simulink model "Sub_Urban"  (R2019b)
settings: Solver=FixedStepAuto  StartTime=0.0  StopTime=3600*24  FixedStep=Tstep  MaxStep=1800  RelTol=1e-3
InitFcn:
  | load('network_parameters')
  | Vnom=400/sqrt(3);
  | Tstep=30*60;
  | MV_LV_transf=0;
StopFcn:
  | run('Simulink_Data.m')
undefined symbols (not defined in the file or in its folder): C_xlpe_185_90, D11, Delta, L_2x16mm, L_2x22mm, L_4x100mm, L_4x16mm, L_4x22mm, L_4x50mm, L_xlpe_185_90, LC, Line_length, R_2x16mm, R_2x22mm, R_4x100mm, R_4x16mm, R_4x22mm, R_4x50mm, R_xlpe_185_90, Source_Voltage
libraries: myLibrary x125, powerlib x89
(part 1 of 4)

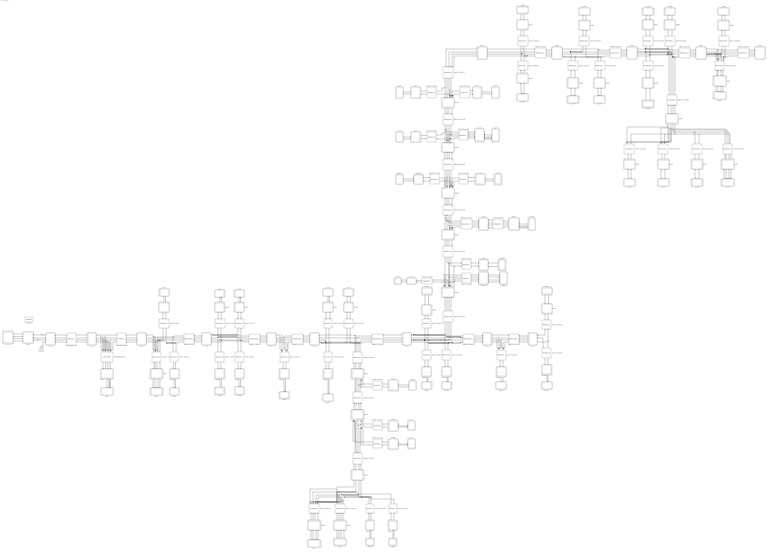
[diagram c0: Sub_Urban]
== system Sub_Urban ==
  100mm^2 Line 12 : powerlib/Elements/Mutual Inductance  LConnTagsString=a|b|c|L4  RConnTagsString=A|B|C|R4  TypeOfMutual=Generalized mutual inductance  NumberOfWindings=4  SelfImpedance1=[1.1 1.1e-03]  SelfImpedance2=[ 1.1 1.1e-03]  ThreeWindings=on  SelfImpedance3=[ 1.1 1.1e-03]  MutualImpedance=[1.0 1.0e-03]  InductanceMatrix=L_4x100mm*Line_length(13)  ResistanceMatrix=R_4x100mm*Line_length(13)  Measurements=None
  100mm^2 Line 14 : powerlib/Elements/Mutual Inductance  LConnTagsString=a|b|c|L4  RConnTagsString=A|B|C|R4  TypeOfMutual=Generalized mutual inductance  NumberOfWindings=4  SelfImpedance1=[1.1 1.1e-03]  SelfImpedance2=[ 1.1 1.1e-03]  ThreeWindings=on  SelfImpedance3=[ 1.1 1.1e-03]  MutualImpedance=[1.0 1.0e-03]  InductanceMatrix=L_4x100mm*Line_length(15)  ResistanceMatrix=R_4x100mm*Line_length(15)  Measurements=None
  100mm^2 Line 18 : powerlib/Elements/Mutual Inductance  LConnTagsString=a|b|c|L4  RConnTagsString=A|B|C|R4  TypeOfMutual=Generalized mutual inductance  NumberOfWindings=4  SelfImpedance1=[1.1 1.1e-03]  SelfImpedance2=[ 1.1 1.1e-03]  ThreeWindings=on  SelfImpedance3=[ 1.1 1.1e-03]  MutualImpedance=[1.0 1.0e-03]  InductanceMatrix=L_4x100mm*Line_length(19)  ResistanceMatrix=R_4x100mm*Line_length(19)  Measurements=None
  100mm^2 Line 20 : powerlib/Elements/Mutual Inductance  LConnTagsString=a|b|c|L4  RConnTagsString=A|B|C|R4  TypeOfMutual=Generalized mutual inductance  NumberOfWindings=4  SelfImpedance1=[1.1 1.1e-03]  SelfImpedance2=[ 1.1 1.1e-03]  ThreeWindings=on  SelfImpedance3=[ 1.1 1.1e-03]  MutualImpedance=[1.0 1.0e-03]  InductanceMatrix=L_4x100mm*Line_length(21)  ResistanceMatrix=R_4x100mm*Line_length(21)  Measurements=None
  100mm^2 Line 23 : powerlib/Elements/Mutual Inductance  LConnTagsString=a|b|c|L4  RConnTagsString=A|B|C|R4  TypeOfMutual=Generalized mutual inductance  NumberOfWindings=4  SelfImpedance1=[1.1 1.1e-03]  SelfImpedance2=[ 1.1 1.1e-03]  ThreeWindings=on  SelfImpedance3=[ 1.1 1.1e-03]  MutualImpedance=[1.0 1.0e-03]  InductanceMatrix=L_4x100mm*Line_length(24)  ResistanceMatrix=R_4x100mm*Line_length(24)  Measurements=None
  100mm^2 Line 28 : powerlib/Elements/Mutual Inductance  LConnTagsString=a|b|c|L4  RConnTagsString=A|B|C|R4  TypeOfMutual=Generalized mutual inductance  NumberOfWindings=4  SelfImpedance1=[1.1 1.1e-03]  SelfImpedance2=[ 1.1 1.1e-03]  ThreeWindings=on  SelfImpedance3=[ 1.1 1.1e-03]  MutualImpedance=[1.0 1.0e-03]  InductanceMatrix=L_4x100mm*Line_length(29)  ResistanceMatrix=R_4x100mm*Line_length(29)  Measurements=None
  100mm^2 Line 29 : powerlib/Elements/Mutual Inductance  LConnTagsString=a|b|c|L4  RConnTagsString=A|B|C|R4  TypeOfMutual=Generalized mutual inductance  NumberOfWindings=4  SelfImpedance1=[1.1 1.1e-03]  SelfImpedance2=[ 1.1 1.1e-03]  ThreeWindings=on  SelfImpedance3=[ 1.1 1.1e-03]  MutualImpedance=[1.0 1.0e-03]  InductanceMatrix=L_4x100mm*Line_length(30)  ResistanceMatrix=R_4x100mm*Line_length(30)  Measurements=None
  100mm^2 Line 31 : powerlib/Elements/Mutual Inductance  LConnTagsString=a|b|c|L4  RConnTagsString=A|B|C|R4  TypeOfMutual=Generalized mutual inductance  NumberOfWindings=4  SelfImpedance1=[1.1 1.1e-03]  SelfImpedance2=[ 1.1 1.1e-03]  ThreeWindings=on  SelfImpedance3=[ 1.1 1.1e-03]  MutualImpedance=[1.0 1.0e-03]  InductanceMatrix=L_4x100mm*Line_length(32)  ResistanceMatrix=R_4x100mm*Line_length(32)  Measurements=None
  100mm^2 Line 37 : powerlib/Elements/Mutual Inductance  LConnTagsString=a|b|c|L4  RConnTagsString=A|B|C|R4  TypeOfMutual=Generalized mutual inductance  NumberOfWindings=4  SelfImpedance1=[1.1 1.1e-03]  SelfImpedance2=[ 1.1 1.1e-03]  ThreeWindings=on  SelfImpedance3=[ 1.1 1.1e-03]  MutualImpedance=[1.0 1.0e-03]  InductanceMatrix=L_4x100mm*Line_length(38)  ResistanceMatrix=R_4x100mm*Line_length(38)  Measurements=None
  100mm^2 Line 41 : powerlib/Elements/Mutual Inductance  LConnTagsString=a|b|c|L4  RConnTagsString=A|B|C|R4  TypeOfMutual=Generalized mutual inductance  NumberOfWindings=4  SelfImpedance1=[1.1 1.1e-03]  SelfImpedance2=[ 1.1 1.1e-03]  ThreeWindings=on  SelfImpedance3=[ 1.1 1.1e-03]  MutualImpedance=[1.0 1.0e-03]  InductanceMatrix=L_4x100mm*Line_length(42)  ResistanceMatrix=R_4x100mm*Line_length(42)  Measurements=None
  100mm^2 Line 42 : powerlib/Elements/Mutual Inductance  LConnTagsString=a|b|c|L4  RConnTagsString=A|B|C|R4  TypeOfMutual=Generalized mutual inductance  NumberOfWindings=4  SelfImpedance1=[1.1 1.1e-03]  SelfImpedance2=[ 1.1 1.1e-03]  ThreeWindings=on  SelfImpedance3=[ 1.1 1.1e-03]  MutualImpedance=[1.0 1.0e-03]  InductanceMatrix=L_4x100mm*Line_length(43)  ResistanceMatrix=R_4x100mm*Line_length(43)  Measurements=None
  100mm^2 Line 44 : powerlib/Elements/Mutual Inductance  LConnTagsString=a|b|c|L4  RConnTagsString=A|B|C|R4  TypeOfMutual=Generalized mutual inductance  NumberOfWindings=4  SelfImpedance1=[1.1 1.1e-03]  SelfImpedance2=[ 1.1 1.1e-03]  ThreeWindings=on  SelfImpedance3=[ 1.1 1.1e-03]  MutualImpedance=[1.0 1.0e-03]  InductanceMatrix=L_4x100mm*Line_length(45)  ResistanceMatrix=R_4x100mm*Line_length(45)  Measurements=None
  100mm^2 Line 47 : powerlib/Elements/Mutual Inductance  LConnTagsString=a|b|c|L4  RConnTagsString=A|B|C|R4  TypeOfMutual=Generalized mutual inductance  NumberOfWindings=4  SelfImpedance1=[1.1 1.1e-03]  SelfImpedance2=[ 1.1 1.1e-03]  ThreeWindings=on  SelfImpedance3=[ 1.1 1.1e-03]  MutualImpedance=[1.0 1.0e-03]  InductanceMatrix=L_4x100mm*Line_length(48)  ResistanceMatrix=R_4x100mm*Line_length(48)  Measurements=None
  100mm^2 Line 50 : powerlib/Elements/Mutual Inductance  LConnTagsString=a|b|c|L4  RConnTagsString=A|B|C|R4  TypeOfMutual=Generalized mutual inductance  NumberOfWindings=4  SelfImpedance1=[1.1 1.1e-03]  SelfImpedance2=[ 1.1 1.1e-03]  ThreeWindings=on  SelfImpedance3=[ 1.1 1.1e-03]  MutualImpedance=[1.0 1.0e-03]  InductanceMatrix=L_4x100mm*Line_length(51)  ResistanceMatrix=R_4x100mm*Line_length(51)  Measurements=None
  100mm^2 Line 68 : powerlib/Elements/Mutual Inductance  LConnTagsString=a|b|c|L4  RConnTagsString=A|B|C|R4  TypeOfMutual=Generalized mutual inductance  NumberOfWindings=4  SelfImpedance1=[1.1 1.1e-03]  SelfImpedance2=[ 1.1 1.1e-03]  ThreeWindings=on  SelfImpedance3=[ 1.1 1.1e-03]  MutualImpedance=[1.0 1.0e-03]  InductanceMatrix=L_4x100mm*Line_length(69)  ResistanceMatrix=R_4x100mm*Line_length(69)  Measurements=None
  100mm^2 Line 7 : powerlib/Elements/Mutual Inductance  LConnTagsString=a|b|c|L4  RConnTagsString=A|B|C|R4  TypeOfMutual=Generalized mutual inductance  NumberOfWindings=4  SelfImpedance1=[1.1 1.1e-03]  SelfImpedance2=[ 1.1 1.1e-03]  ThreeWindings=on  SelfImpedance3=[ 1.1 1.1e-03]  MutualImpedance=[1.0 1.0e-03]  InductanceMatrix=L_4x100mm*Line_length(8)  ResistanceMatrix=R_4x100mm*Line_length(8)  Measurements=None
  16mm^2 Line 24 : powerlib/Elements/Mutual Inductance  LConnTagsString=a|b|c|L4  RConnTagsString=A|B|C|R4  TypeOfMutual=Generalized mutual inductance  NumberOfWindings=4  SelfImpedance1=[1.1 1.1e-03]  SelfImpedance2=[ 1.1 1.1e-03]  ThreeWindings=on  SelfImpedance3=[ 1.1 1.1e-03]  MutualImpedance=[1.0 1.0e-03]  InductanceMatrix=L_4x16mm*Line_length(25)  ResistanceMatrix=R_4x16mm*Line_length(25)  Measurements=None
  16mm^2 Line 25 : powerlib/Elements/Mutual Inductance  LConnTagsString=a|b|c|L4  RConnTagsString=A|B|C|R4  TypeOfMutual=Generalized mutual inductance  NumberOfWindings=4  SelfImpedance1=[1.1 1.1e-03]  SelfImpedance2=[ 1.1 1.1e-03]  ThreeWindings=on  SelfImpedance3=[ 1.1 1.1e-03]  MutualImpedance=[1.0 1.0e-03]  InductanceMatrix=L_4x16mm*Line_length(26)  ResistanceMatrix=R_4x16mm*Line_length(26)  Measurements=None
  16mm^2 Line 34 : powerlib/Elements/Mutual Inductance  LConnTagsString=a|b  RConnTagsString=A|B  TypeOfMutual=Generalized mutual inductance  NumberOfWindings=2  SelfImpedance1=[1.1 1.1e-03]  SelfImpedance2=[ 1.1 1.1e-03]  ThreeWindings=on  SelfImpedance3=[ 1.1 1.1e-03]  MutualImpedance=[1.0 1.0e-03]  InductanceMatrix=L_2x16mm*Line_length(35)  ResistanceMatrix=R_2x16mm*Line_length(35)  Measurements=None
  16mm^2 Line 62 : powerlib/Elements/Mutual Inductance  LConnTagsString=a|b|c|L4  RConnTagsString=A|B|C|R4  TypeOfMutual=Generalized mutual inductance  NumberOfWindings=4  SelfImpedance1=[1.1 1.1e-03]  SelfImpedance2=[ 1.1 1.1e-03]  ThreeWindings=on  SelfImpedance3=[ 1.1 1.1e-03]  MutualImpedance=[1.0 1.0e-03]  InductanceMatrix=L_4x16mm*Line_length(63)  ResistanceMatrix=R_4x16mm*Line_length(63)  Measurements=None
  16mm^2 Line 8 : powerlib/Elements/Mutual Inductance  LConnTagsString=a|b  RConnTagsString=A|B  TypeOfMutual=Generalized mutual inductance  NumberOfWindings=2  SelfImpedance1=[1.1 1.1e-03]  SelfImpedance2=[ 1.1 1.1e-03]  ThreeWindings=on  SelfImpedance3=[ 1.1 1.1e-03]  MutualImpedance=[1.0 1.0e-03]  InductanceMatrix=L_2x16mm*Line_length(9)  ResistanceMatrix=R_2x16mm*Line_length(9)  Measurements=None
  22mm^2 Line 10 : powerlib/Elements/Mutual Inductance  LConnTagsString=a|b  RConnTagsString=A|B  TypeOfMutual=Generalized mutual inductance  NumberOfWindings=2  SelfImpedance1=[1.1 1.1e-03]  SelfImpedance2=[ 1.1 1.1e-03]  ThreeWindings=on  SelfImpedance3=[ 1.1 1.1e-03]  MutualImpedance=[1.0 1.0e-03]  InductanceMatrix=L_2x22mm*Line_length(11)  ResistanceMatrix=R_2x22mm*Line_length(11)  Measurements=None
  22mm^2 Line 11 : powerlib/Elements/Mutual Inductance  LConnTagsString=a|b  RConnTagsString=A|B  TypeOfMutual=Generalized mutual inductance  NumberOfWindings=2  SelfImpedance1=[1.1 1.1e-03]  SelfImpedance2=[ 1.1 1.1e-03]  ThreeWindings=on  SelfImpedance3=[ 1.1 1.1e-03]  MutualImpedance=[1.0 1.0e-03]  InductanceMatrix=L_2x22mm*Line_length(12)  ResistanceMatrix=R_2x22mm*Line_length(12)  Measurements=None
  22mm^2 Line 13 : powerlib/Elements/Mutual Inductance  LConnTagsString=a|b  RConnTagsString=A|B  TypeOfMutual=Generalized mutual inductance  NumberOfWindings=2  SelfImpedance1=[1.1 1.1e-03]  SelfImpedance2=[ 1.1 1.1e-03]  ThreeWindings=on  SelfImpedance3=[ 1.1 1.1e-03]  MutualImpedance=[1.0 1.0e-03]  InductanceMatrix=L_2x22mm*Line_length(14)  ResistanceMatrix=R_2x22mm*Line_length(14)  Measurements=None
  22mm^2 Line 15 : powerlib/Elements/Mutual Inductance  LConnTagsString=a|b  RConnTagsString=A|B  TypeOfMutual=Generalized mutual inductance  NumberOfWindings=2  SelfImpedance1=[1.1 1.1e-03]  SelfImpedance2=[ 1.1 1.1e-03]  ThreeWindings=on  SelfImpedance3=[ 1.1 1.1e-03]  MutualImpedance=[1.0 1.0e-03]  InductanceMatrix=L_2x22mm*Line_length(16)  ResistanceMatrix=R_2x22mm*Line_length(16)  Measurements=None
  22mm^2 Line 16 : powerlib/Elements/Mutual Inductance  LConnTagsString=a|b  RConnTagsString=A|B  TypeOfMutual=Generalized mutual inductance  NumberOfWindings=2  SelfImpedance1=[1.1 1.1e-03]  SelfImpedance2=[ 1.1 1.1e-03]  ThreeWindings=on  SelfImpedance3=[ 1.1 1.1e-03]  MutualImpedance=[1.0 1.0e-03]  InductanceMatrix=L_2x22mm*Line_length(17)  ResistanceMatrix=R_2x22mm*Line_length(17)  Measurements=None
  22mm^2 Line 17 : powerlib/Elements/Mutual Inductance  LConnTagsString=a|b  RConnTagsString=A|B  TypeOfMutual=Generalized mutual inductance  NumberOfWindings=2  SelfImpedance1=[1.1 1.1e-03]  SelfImpedance2=[ 1.1 1.1e-03]  ThreeWindings=on  SelfImpedance3=[ 1.1 1.1e-03]  MutualImpedance=[1.0 1.0e-03]  InductanceMatrix=L_2x22mm*Line_length(18)  ResistanceMatrix=R_2x22mm*Line_length(18)  Measurements=None
  22mm^2 Line 19 : powerlib/Elements/Mutual Inductance  LConnTagsString=a|b  RConnTagsString=A|B  TypeOfMutual=Generalized mutual inductance  NumberOfWindings=2  SelfImpedance1=[1.1 1.1e-03]  SelfImpedance2=[ 1.1 1.1e-03]  ThreeWindings=on  SelfImpedance3=[ 1.1 1.1e-03]  MutualImpedance=[1.0 1.0e-03]  InductanceMatrix=L_2x22mm*Line_length(20)  ResistanceMatrix=R_2x22mm*Line_length(20)  Measurements=None
  22mm^2 Line 21 : powerlib/Elements/Mutual Inductance  LConnTagsString=a|b  RConnTagsString=A|B  TypeOfMutual=Generalized mutual inductance  NumberOfWindings=2  SelfImpedance1=[1.1 1.1e-03]  SelfImpedance2=[ 1.1 1.1e-03]  ThreeWindings=on  SelfImpedance3=[ 1.1 1.1e-03]  MutualImpedance=[1.0 1.0e-03]  InductanceMatrix=L_2x22mm*Line_length(22)  ResistanceMatrix=R_2x22mm*Line_length(22)  Measurements=None
  22mm^2 Line 22 : powerlib/Elements/Mutual Inductance  LConnTagsString=a|b  RConnTagsString=A|B  TypeOfMutual=Generalized mutual inductance  NumberOfWindings=2  SelfImpedance1=[1.1 1.1e-03]  SelfImpedance2=[ 1.1 1.1e-03]  ThreeWindings=on  SelfImpedance3=[ 1.1 1.1e-03]  MutualImpedance=[1.0 1.0e-03]  InductanceMatrix=L_2x22mm*Line_length(23)  ResistanceMatrix=R_2x22mm*Line_length(23)  Measurements=None
  22mm^2 Line 26 : powerlib/Elements/Mutual Inductance  LConnTagsString=a|b  RConnTagsString=A|B  TypeOfMutual=Generalized mutual inductance  NumberOfWindings=2  SelfImpedance1=[1.1 1.1e-03]  SelfImpedance2=[ 1.1 1.1e-03]  ThreeWindings=on  SelfImpedance3=[ 1.1 1.1e-03]  MutualImpedance=[1.0 1.0e-03]  InductanceMatrix=L_2x22mm*Line_length(27)  ResistanceMatrix=R_2x22mm*Line_length(27)  Measurements=None
  22mm^2 Line 27 : powerlib/Elements/Mutual Inductance  LConnTagsString=a|b  RConnTagsString=A|B  TypeOfMutual=Generalized mutual inductance  NumberOfWindings=2  SelfImpedance1=[1.1 1.1e-03]  SelfImpedance2=[ 1.1 1.1e-03]  ThreeWindings=on  SelfImpedance3=[ 1.1 1.1e-03]  MutualImpedance=[1.0 1.0e-03]  InductanceMatrix=L_2x22mm*Line_length(28)  ResistanceMatrix=R_2x22mm*Line_length(28)  Measurements=None
  22mm^2 Line 30 : powerlib/Elements/Mutual Inductance  LConnTagsString=a|b  RConnTagsString=A|B  TypeOfMutual=Generalized mutual inductance  NumberOfWindings=2  SelfImpedance1=[1.1 1.1e-03]  SelfImpedance2=[ 1.1 1.1e-03]  ThreeWindings=on  SelfImpedance3=[ 1.1 1.1e-03]  MutualImpedance=[1.0 1.0e-03]  InductanceMatrix=L_2x22mm*Line_length(31)  ResistanceMatrix=R_2x22mm*Line_length(31)  Measurements=None
  22mm^2 Line 32 : powerlib/Elements/Mutual Inductance  LConnTagsString=a|b  RConnTagsString=A|B  TypeOfMutual=Generalized mutual inductance  NumberOfWindings=2  SelfImpedance1=[1.1 1.1e-03]  SelfImpedance2=[ 1.1 1.1e-03]  ThreeWindings=on  SelfImpedance3=[ 1.1 1.1e-03]  MutualImpedance=[1.0 1.0e-03]  InductanceMatrix=L_2x22mm*Line_length(33)  ResistanceMatrix=R_2x22mm*Line_length(33)  Measurements=None
  22mm^2 Line 33 : powerlib/Elements/Mutual Inductance  LConnTagsString=a|b  RConnTagsString=A|B  TypeOfMutual=Generalized mutual inductance  NumberOfWindings=2  SelfImpedance1=[1.1 1.1e-03]  SelfImpedance2=[ 1.1 1.1e-03]  ThreeWindings=on  SelfImpedance3=[ 1.1 1.1e-03]  MutualImpedance=[1.0 1.0e-03]  InductanceMatrix=L_2x22mm*Line_length(34)  ResistanceMatrix=R_2x22mm*Line_length(34)  Measurements=None
  22mm^2 Line 35 : powerlib/Elements/Mutual Inductance  LConnTagsString=a|b  RConnTagsString=A|B  TypeOfMutual=Generalized mutual inductance  NumberOfWindings=2  SelfImpedance1=[1.1 1.1e-03]  SelfImpedance2=[ 1.1 1.1e-03]  ThreeWindings=on  SelfImpedance3=[ 1.1 1.1e-03]  MutualImpedance=[1.0 1.0e-03]  InductanceMatrix=L_2x22mm*Line_length(36)  ResistanceMatrix=R_2x22mm*Line_length(36)  Measurements=None
  22mm^2 Line 36 : powerlib/Elements/Mutual Inductance  LConnTagsString=a|b  RConnTagsString=A|B  TypeOfMutual=Generalized mutual inductance  NumberOfWindings=2  SelfImpedance1=[1.1 1.1e-03]  SelfImpedance2=[ 1.1 1.1e-03]  ThreeWindings=on  SelfImpedance3=[ 1.1 1.1e-03]  MutualImpedance=[1.0 1.0e-03]  InductanceMatrix=L_2x22mm*Line_length(37)  ResistanceMatrix=R_2x22mm*Line_length(37)  Measurements=None
  22mm^2 Line 38 : powerlib/Elements/Mutual Inductance  LConnTagsString=a|b|c|L4  RConnTagsString=A|B|C|R4  TypeOfMutual=Generalized mutual inductance  NumberOfWindings=4  SelfImpedance1=[1.1 1.1e-03]  SelfImpedance2=[ 1.1 1.1e-03]  ThreeWindings=on  SelfImpedance3=[ 1.1 1.1e-03]  MutualImpedance=[1.0 1.0e-03]  InductanceMatrix=L_4x22mm*Line_length(39)  ResistanceMatrix=R_4x22mm*Line_length(39)  Measurements=None
  22mm^2 Line 39 : powerlib/Elements/Mutual Inductance  LConnTagsString=a|b  RConnTagsString=A|B  TypeOfMutual=Generalized mutual inductance  NumberOfWindings=2  SelfImpedance1=[1.1 1.1e-03]  SelfImpedance2=[ 1.1 1.1e-03]  ThreeWindings=on  SelfImpedance3=[ 1.1 1.1e-03]  MutualImpedance=[1.0 1.0e-03]  InductanceMatrix=L_2x22mm*Line_length(40)  ResistanceMatrix=R_2x22mm*Line_length(40)  Measurements=None
  22mm^2 Line 4 : powerlib/Elements/Mutual Inductance  LConnTagsString=a|b|c|L4  RConnTagsString=A|B|C|R4  TypeOfMutual=Generalized mutual inductance  NumberOfWindings=4  SelfImpedance1=[1.1 1.1e-03]  SelfImpedance2=[ 1.1 1.1e-03]  ThreeWindings=on  SelfImpedance3=[ 1.1 1.1e-03]  MutualImpedance=[1.0 1.0e-03]  InductanceMatrix=L_4x22mm*Line_length(5)  ResistanceMatrix=R_4x22mm*Line_length(5)  Measurements=None
  22mm^2 Line 40 : powerlib/Elements/Mutual Inductance  LConnTagsString=a|b  RConnTagsString=A|B  TypeOfMutual=Generalized mutual inductance  NumberOfWindings=2  SelfImpedance1=[1.1 1.1e-03]  SelfImpedance2=[ 1.1 1.1e-03]  ThreeWindings=on  SelfImpedance3=[ 1.1 1.1e-03]  MutualImpedance=[1.0 1.0e-03]  InductanceMatrix=L_2x22mm*Line_length(41)  ResistanceMatrix=R_2x22mm*Line_length(41)  Measurements=None
  22mm^2 Line 43 : powerlib/Elements/Mutual Inductance  LConnTagsString=a|b|c|L4  RConnTagsString=A|B|C|R4  TypeOfMutual=Generalized mutual inductance  NumberOfWindings=4  SelfImpedance1=[1.1 1.1e-03]  SelfImpedance2=[ 1.1 1.1e-03]  ThreeWindings=on  SelfImpedance3=[ 1.1 1.1e-03]  MutualImpedance=[1.0 1.0e-03]  InductanceMatrix=L_4x22mm*Line_length(44)  ResistanceMatrix=R_4x22mm*Line_length(44)  Measurements=None
  22mm^2 Line 45 : powerlib/Elements/Mutual Inductance  LConnTagsString=a|b  RConnTagsString=A|B  TypeOfMutual=Generalized mutual inductance  NumberOfWindings=2  SelfImpedance1=[1.1 1.1e-03]  SelfImpedance2=[ 1.1 1.1e-03]  ThreeWindings=on  SelfImpedance3=[ 1.1 1.1e-03]  MutualImpedance=[1.0 1.0e-03]  InductanceMatrix=L_2x22mm*Line_length(46)  ResistanceMatrix=R_2x22mm*Line_length(46)  Measurements=None
  22mm^2 Line 46 : powerlib/Elements/Mutual Inductance  LConnTagsString=a|b  RConnTagsString=A|B  TypeOfMutual=Generalized mutual inductance  NumberOfWindings=2  SelfImpedance1=[1.1 1.1e-03]  SelfImpedance2=[ 1.1 1.1e-03]  ThreeWindings=on  SelfImpedance3=[ 1.1 1.1e-03]  MutualImpedance=[1.0 1.0e-03]  InductanceMatrix=L_2x22mm*Line_length(47)  ResistanceMatrix=R_2x22mm*Line_length(47)  Measurements=None
  22mm^2 Line 48 : powerlib/Elements/Mutual Inductance  LConnTagsString=a|b|c|L4  RConnTagsString=A|B|C|R4  TypeOfMutual=Generalized mutual inductance  NumberOfWindings=4  SelfImpedance1=[1.1 1.1e-03]  SelfImpedance2=[ 1.1 1.1e-03]  ThreeWindings=on  SelfImpedance3=[ 1.1 1.1e-03]  MutualImpedance=[1.0 1.0e-03]  InductanceMatrix=L_4x22mm*Line_length(49)  ResistanceMatrix=R_4x22mm*Line_length(49)  Measurements=None
  22mm^2 Line 49 : powerlib/Elements/Mutual Inductance  LConnTagsString=a|b  RConnTagsString=A|B  TypeOfMutual=Generalized mutual inductance  NumberOfWindings=2  SelfImpedance1=[1.1 1.1e-03]  SelfImpedance2=[ 1.1 1.1e-03]  ThreeWindings=on  SelfImpedance3=[ 1.1 1.1e-03]  MutualImpedance=[1.0 1.0e-03]  InductanceMatrix=L_2x22mm*Line_length(50)  ResistanceMatrix=R_2x22mm*Line_length(50)  Measurements=None
  22mm^2 Line 5 : powerlib/Elements/Mutual Inductance  LConnTagsString=a|b  RConnTagsString=A|B  TypeOfMutual=Generalized mutual inductance  NumberOfWindings=2  SelfImpedance1=[1.1 1.1e-03]  SelfImpedance2=[ 1.1 1.1e-03]  ThreeWindings=on  SelfImpedance3=[ 1.1 1.1e-03]  MutualImpedance=[1.0 1.0e-03]  InductanceMatrix=L_2x22mm*Line_length(6)  ResistanceMatrix=R_2x22mm*Line_length(6)  Measurements=None
  22mm^2 Line 51 : powerlib/Elements/Mutual Inductance  LConnTagsString=a|b  RConnTagsString=A|B  TypeOfMutual=Generalized mutual inductance  NumberOfWindings=2  SelfImpedance1=[1.1 1.1e-03]  SelfImpedance2=[ 1.1 1.1e-03]  ThreeWindings=on  SelfImpedance3=[ 1.1 1.1e-03]  MutualImpedance=[1.0 1.0e-03]  InductanceMatrix=L_2x22mm*Line_length(52)  ResistanceMatrix=R_2x22mm*Line_length(52)  Measurements=None
  22mm^2 Line 52 : powerlib/Elements/Mutual Inductance  LConnTagsString=a|b  RConnTagsString=A|B  TypeOfMutual=Generalized mutual inductance  NumberOfWindings=2  SelfImpedance1=[1.1 1.1e-03]  SelfImpedance2=[ 1.1 1.1e-03]  ThreeWindings=on  SelfImpedance3=[ 1.1 1.1e-03]  MutualImpedance=[1.0 1.0e-03]  InductanceMatrix=L_2x22mm*Line_length(53)  ResistanceMatrix=R_2x22mm*Line_length(53)  Measurements=None
  22mm^2 Line 54 : powerlib/Elements/Mutual Inductance  LConnTagsString=a|b  RConnTagsString=A|B  TypeOfMutual=Generalized mutual inductance  NumberOfWindings=2  SelfImpedance1=[1.1 1.1e-03]  SelfImpedance2=[ 1.1 1.1e-03]  ThreeWindings=on  SelfImpedance3=[ 1.1 1.1e-03]  MutualImpedance=[1.0 1.0e-03]  InductanceMatrix=L_2x22mm*Line_length(55)  ResistanceMatrix=R_2x22mm*Line_length(55)  Measurements=None
  22mm^2 Line 55 : powerlib/Elements/Mutual Inductance  LConnTagsString=a|b  RConnTagsString=A|B  TypeOfMutual=Generalized mutual inductance  NumberOfWindings=2  SelfImpedance1=[1.1 1.1e-03]  SelfImpedance2=[ 1.1 1.1e-03]  ThreeWindings=on  SelfImpedance3=[ 1.1 1.1e-03]  MutualImpedance=[1.0 1.0e-03]  InductanceMatrix=L_2x22mm*Line_length(56)  ResistanceMatrix=R_2x22mm*Line_length(56)  Measurements=None
  22mm^2 Line 57 : powerlib/Elements/Mutual Inductance  LConnTagsString=a|b  RConnTagsString=A|B  TypeOfMutual=Generalized mutual inductance  NumberOfWindings=2  SelfImpedance1=[1.1 1.1e-03]  SelfImpedance2=[ 1.1 1.1e-03]  ThreeWindings=on  SelfImpedance3=[ 1.1 1.1e-03]  MutualImpedance=[1.0 1.0e-03]  InductanceMatrix=L_2x22mm*Line_length(58)  ResistanceMatrix=R_2x22mm*Line_length(58)  Measurements=None
  22mm^2 Line 58 : powerlib/Elements/Mutual Inductance  LConnTagsString=a|b  RConnTagsString=A|B  TypeOfMutual=Generalized mutual inductance  NumberOfWindings=2  SelfImpedance1=[1.1 1.1e-03]  SelfImpedance2=[ 1.1 1.1e-03]  ThreeWindings=on  SelfImpedance3=[ 1.1 1.1e-03]  MutualImpedance=[1.0 1.0e-03]  InductanceMatrix=L_2x22mm*Line_length(59)  ResistanceMatrix=R_2x22mm*Line_length(59)  Measurements=None
  22mm^2 Line 59 : powerlib/Elements/Mutual Inductance  LConnTagsString=a|b  RConnTagsString=A|B  TypeOfMutual=Generalized mutual inductance  NumberOfWindings=2  SelfImpedance1=[1.1 1.1e-03]  SelfImpedance2=[ 1.1 1.1e-03]  ThreeWindings=on  SelfImpedance3=[ 1.1 1.1e-03]  MutualImpedance=[1.0 1.0e-03]  InductanceMatrix=L_2x22mm*Line_length(60)  ResistanceMatrix=R_2x22mm*Line_length(60)  Measurements=None
  22mm^2 Line 6 : powerlib/Elements/Mutual Inductance  LConnTagsString=a|b  RConnTagsString=A|B  TypeOfMutual=Generalized mutual inductance  NumberOfWindings=2  SelfImpedance1=[1.1 1.1e-03]  SelfImpedance2=[ 1.1 1.1e-03]  ThreeWindings=on  SelfImpedance3=[ 1.1 1.1e-03]  MutualImpedance=[1.0 1.0e-03]  InductanceMatrix=L_2x22mm*Line_length(7)  ResistanceMatrix=R_2x22mm*Line_length(7)  Measurements=None
  22mm^2 Line 63 : powerlib/Elements/Mutual Inductance  LConnTagsString=a|b  RConnTagsString=A|B  TypeOfMutual=Generalized mutual inductance  NumberOfWindings=2  SelfImpedance1=[1.1 1.1e-03]  SelfImpedance2=[ 1.1 1.1e-03]  ThreeWindings=on  SelfImpedance3=[ 1.1 1.1e-03]  MutualImpedance=[1.0 1.0e-03]  InductanceMatrix=L_2x22mm*Line_length(64)  ResistanceMatrix=R_2x22mm*Line_length(64)  Measurements=None
  22mm^2 Line 65 : powerlib/Elements/Mutual Inductance  LConnTagsString=a|b  RConnTagsString=A|B  TypeOfMutual=Generalized mutual inductance  NumberOfWindings=2  SelfImpedance1=[1.1 1.1e-03]  SelfImpedance2=[ 1.1 1.1e-03]  ThreeWindings=on  SelfImpedance3=[ 1.1 1.1e-03]  MutualImpedance=[1.0 1.0e-03]  InductanceMatrix=L_2x22mm*Line_length(66)  ResistanceMatrix=R_2x22mm*Line_length(66)  Measurements=None
  22mm^2 Line 66 : powerlib/Elements/Mutual Inductance  LConnTagsString=a|b  RConnTagsString=A|B  TypeOfMutual=Generalized mutual inductance  NumberOfWindings=2  SelfImpedance1=[1.1 1.1e-03]  SelfImpedance2=[ 1.1 1.1e-03]  ThreeWindings=on  SelfImpedance3=[ 1.1 1.1e-03]  MutualImpedance=[1.0 1.0e-03]  InductanceMatrix=L_2x22mm*Line_length(67)  ResistanceMatrix=R_2x22mm*Line_length(67)  Measurements=None
  22mm^2 Line 67 : powerlib/Elements/Mutual Inductance  LConnTagsString=a|b  RConnTagsString=A|B  TypeOfMutual=Generalized mutual inductance  NumberOfWindings=2  SelfImpedance1=[1.1 1.1e-03]  SelfImpedance2=[ 1.1 1.1e-03]  ThreeWindings=on  SelfImpedance3=[ 1.1 1.1e-03]  MutualImpedance=[1.0 1.0e-03]  InductanceMatrix=L_2x22mm*Line_length(68)  ResistanceMatrix=R_2x22mm*Line_length(68)  Measurements=None
  22mm^2 Line 69 : powerlib/Elements/Mutual Inductance  LConnTagsString=a|b  RConnTagsString=A|B  TypeOfMutual=Generalized mutual inductance  NumberOfWindings=2  SelfImpedance1=[1.1 1.1e-03]  SelfImpedance2=[ 1.1 1.1e-03]  ThreeWindings=on  SelfImpedance3=[ 1.1 1.1e-03]  MutualImpedance=[1.0 1.0e-03]  InductanceMatrix=L_2x22mm*Line_length(70)  ResistanceMatrix=R_2x22mm*Line_length(70)  Measurements=None
  22mm^2 Line 70 : powerlib/Elements/Mutual Inductance  LConnTagsString=a|b  RConnTagsString=A|B  TypeOfMutual=Generalized mutual inductance  NumberOfWindings=2  SelfImpedance1=[1.1 1.1e-03]  SelfImpedance2=[ 1.1 1.1e-03]  ThreeWindings=on  SelfImpedance3=[ 1.1 1.1e-03]  MutualImpedance=[1.0 1.0e-03]  InductanceMatrix=L_2x22mm*Line_length(71)  ResistanceMatrix=R_2x22mm*Line_length(71)  Measurements=None
  22mm^2 Line 71 : powerlib/Elements/Mutual Inductance  LConnTagsString=a|b  RConnTagsString=A|B  TypeOfMutual=Generalized mutual inductance  NumberOfWindings=2  SelfImpedance1=[1.1 1.1e-03]  SelfImpedance2=[ 1.1 1.1e-03]  ThreeWindings=on  SelfImpedance3=[ 1.1 1.1e-03]  MutualImpedance=[1.0 1.0e-03]  InductanceMatrix=L_2x22mm*Line_length(72)  ResistanceMatrix=R_2x22mm*Line_length(72)  Measurements=None
  22mm^2 Line 72 : powerlib/Elements/Mutual Inductance  LConnTagsString=a|b|c|L4  RConnTagsString=A|B|C|R4  TypeOfMutual=Generalized mutual inductance  NumberOfWindings=4  SelfImpedance1=[1.1 1.1e-03]  SelfImpedance2=[ 1.1 1.1e-03]  ThreeWindings=on  SelfImpedance3=[ 1.1 1.1e-03]  MutualImpedance=[1.0 1.0e-03]  InductanceMatrix=L_4x22mm*Line_length(73)  ResistanceMatrix=R_4x22mm*Line_length(73)  Measurements=None
  22mm^2 Line 9 : powerlib/Elements/Mutual Inductance  LConnTagsString=a|b  RConnTagsString=A|B  TypeOfMutual=Generalized mutual inductance  NumberOfWindings=2  SelfImpedance1=[1.1 1.1e-03]  SelfImpedance2=[ 1.1 1.1e-03]  ThreeWindings=on  SelfImpedance3=[ 1.1 1.1e-03]  MutualImpedance=[1.0 1.0e-03]  InductanceMatrix=L_2x22mm*Line_length(10)  ResistanceMatrix=R_2x22mm*Line_length(10)  Measurements=None
  50mm^2 Line 53 : powerlib/Elements/Mutual Inductance  LConnTagsString=a|b|c|L4  RConnTagsString=A|B|C|R4  TypeOfMutual=Generalized mutual inductance  NumberOfWindings=4  SelfImpedance1=[1.1 1.1e-03]  SelfImpedance2=[ 1.1 1.1e-03]  ThreeWindings=on  SelfImpedance3=[ 1.1 1.1e-03]  MutualImpedance=[1.0 1.0e-03]  InductanceMatrix=L_4x50mm*Line_length(54)  ResistanceMatrix=R_4x50mm*Line_length(54)  Measurements=None
  50mm^2 Line 56 : powerlib/Elements/Mutual Inductance  LConnTagsString=a|b|c|L4  RConnTagsString=A|B|C|R4  TypeOfMutual=Generalized mutual inductance  NumberOfWindings=4  SelfImpedance1=[1.1 1.1e-03]  SelfImpedance2=[ 1.1 1.1e-03]  ThreeWindings=on  SelfImpedance3=[ 1.1 1.1e-03]  MutualImpedance=[1.0 1.0e-03]  InductanceMatrix=L_4x50mm*Line_length(57)  ResistanceMatrix=R_4x50mm*Line_length(57)  Measurements=None
  50mm^2 Line 60 : powerlib/Elements/Mutual Inductance  LConnTagsString=a|b|c|L4  RConnTagsString=A|B|C|R4  TypeOfMutual=Generalized mutual inductance  NumberOfWindings=4  SelfImpedance1=[1.1 1.1e-03]  SelfImpedance2=[ 1.1 1.1e-03]  ThreeWindings=on  SelfImpedance3=[ 1.1 1.1e-03]  MutualImpedance=[1.0 1.0e-03]  InductanceMatrix=L_4x50mm*Line_length(61)  ResistanceMatrix=R_4x50mm*Line_length(61)  Measurements=None
  50mm^2 Line 61 : powerlib/Elements/Mutual Inductance  LConnTagsString=a|b|c|L4  RConnTagsString=A|B|C|R4  TypeOfMutual=Generalized mutual inductance  NumberOfWindings=4  SelfImpedance1=[1.1 1.1e-03]  SelfImpedance2=[ 1.1 1.1e-03]  ThreeWindings=on  SelfImpedance3=[ 1.1 1.1e-03]  MutualImpedance=[1.0 1.0e-03]  InductanceMatrix=L_4x50mm*Line_length(62)  ResistanceMatrix=R_4x50mm*Line_length(62)  Measurements=None
  50mm^2 Line 64 : powerlib/Elements/Mutual Inductance  LConnTagsString=a|b|c|L4  RConnTagsString=A|B|C|R4  TypeOfMutual=Generalized mutual inductance  NumberOfWindings=4  SelfImpedance1=[1.1 1.1e-03]  SelfImpedance2=[ 1.1 1.1e-03]  ThreeWindings=on  SelfImpedance3=[ 1.1 1.1e-03]  MutualImpedance=[1.0 1.0e-03]  InductanceMatrix=L_4x50mm*Line_length(65)  ResistanceMatrix=R_4x50mm*Line_length(65)  Measurements=None
  Bus1 : Subsystem
  Bus10 : Subsystem  mask{Ph=3, Bus=10, Load=5}
      mask prompts: Ph "Phase [A=1, B=2, C=3]"; Bus "Bus Number"; Load "Load Number"
      mask init:
      | data_V=sprintf('Bus%d',Bus);
      | set_param([gcb '/To Workspace V'],'VariableName',data_V);
      | 
      | data_I=sprintf('I%d',Bus);
      | set_param([gcb '/To Workspace I'],'VariableName',data_I);
      | 
      | data_L=sprintf('Load%d',Load);
      | set_param([gcb '/To Workspace L'],'VariableName',data_L)
  Bus11 : Subsystem  mask{Ph=2, Bus=11, Load=6}
      mask prompts: Ph "Phase [A=1, B=2, C=3]"; Bus "Bus Number"; Load "Load Number"
      mask init:
      | data_V=sprintf('Bus%d',Bus);
      | set_param([gcb '/To Workspace V'],'VariableName',data_V);
      | 
      | data_I=sprintf('I%d',Bus);
      | set_param([gcb '/To Workspace I'],'VariableName',data_I);
      | 
      | data_L=sprintf('Load%d',Load);
      | set_param([gcb '/To Workspace L'],'VariableName',data_L)
  Bus12 : Subsystem  mask{Ph=2, Bus=12, Load=7}
      mask prompts: Ph "Phase [A=1, B=2, C=3]"; Bus "Bus Number"; Load "Load Number"
      mask init:
      | data_V=sprintf('Bus%d',Bus);
      | set_param([gcb '/To Workspace V'],'VariableName',data_V);
      | 
      | data_I=sprintf('I%d',Bus);
      | set_param([gcb '/To Workspace I'],'VariableName',data_I);
      | 
      | data_L=sprintf('Load%d',Load);
      | set_param([gcb '/To Workspace L'],'VariableName',data_L)
  Bus13 : Subsystem  mask{Ph=1, Bus=13, Load=8}
      mask prompts: Ph "Phase [A=1, B=2, C=3]"; Bus "Bus Number"; Load "Load Number"
      mask init:
      | data_V=sprintf('Bus%d',Bus);
      | set_param([gcb '/To Workspace V'],'VariableName',data_V);
      | 
      | data_I=sprintf('I%d',Bus);
      | set_param([gcb '/To Workspace I'],'VariableName',data_I);
      | 
      | data_L=sprintf('Load%d',Load);
      | set_param([gcb '/To Workspace L'],'VariableName',data_L)
  Bus14 : Subsystem  mask{Bus=14}
      mask prompts: Bus "Bus Number"
      mask init:
      | data_V=sprintf('Bus%d',Bus);
      | set_param([gcb '/To Workspace V'],'VariableName',data_V);
      | 
      | data_I=sprintf('I%d',Bus);
      | set_param([gcb '/To Workspace I'],'VariableName',data_I);
  Bus15 : Subsystem  mask{Ph=1, Bus=15, Load=9}
      mask prompts: Ph "Phase [A=1, B=2, C=3]"; Bus "Bus Number"; Load "Load Number"
      mask init:
      | data_V=sprintf('Bus%d',Bus);
      | set_param([gcb '/To Workspace V'],'VariableName',data_V);
      | 
      | data_I=sprintf('I%d',Bus);
      | set_param([gcb '/To Workspace I'],'VariableName',data_I);
      | 
      | data_L=sprintf('Load%d',Load);
      | set_param([gcb '/To Workspace L'],'VariableName',data_L)
  Bus16 : Subsystem  mask{Bus=16}
      mask prompts: Bus "Bus Number"
      mask init:
      | data_V=sprintf('Bus%d',Bus);
      | set_param([gcb '/To Workspace V'],'VariableName',data_V);
      | 
      | data_I=sprintf('I%d',Bus);
      | set_param([gcb '/To Workspace I'],'VariableName',data_I);
  Bus17 : Subsystem  mask{Ph=3, Bus=17, Load=10}
      mask prompts: Ph "Phase [A=1, B=2, C=3]"; Bus "Bus Number"; Load "Load Number"
      mask init:
      | data_V=sprintf('Bus%d',Bus);
      | set_param([gcb '/To Workspace V'],'VariableName',data_V);
      | 
      | data_I=sprintf('I%d',Bus);
      | set_param([gcb '/To Workspace I'],'VariableName',data_I);
      | 
      | data_L=sprintf('Load%d',Load);
      | set_param([gcb '/To Workspace L'],'VariableName',data_L)
  Bus18 : Subsystem  mask{Ph=3, Bus=18, Load=11}
      mask prompts: Ph "Phase [A=1, B=2, C=3]"; Bus "Bus Number"; Load "Load Number"
      mask init:
      | data_V=sprintf('Bus%d',Bus);
      | set_param([gcb '/To Workspace V'],'VariableName',data_V);
      | 
      | data_I=sprintf('I%d',Bus);
      | set_param([gcb '/To Workspace I'],'VariableName',data_I);
      | 
      | data_L=sprintf('Load%d',Load);
      | set_param([gcb '/To Workspace L'],'VariableName',data_L)
  Bus19 : Subsystem  mask{Ph=3, Bus=19, Load=12}
      mask prompts: Ph "Phase [A=1, B=2, C=3]"; Bus "Bus Number"; Load "Load Number"
      mask init:
      | data_V=sprintf('Bus%d',Bus);
      | set_param([gcb '/To Workspace V'],'VariableName',data_V);
      | 
      | data_I=sprintf('I%d',Bus);
      | set_param([gcb '/To Workspace I'],'VariableName',data_I);
      | 
      | data_L=sprintf('Load%d',Load);
      | set_param([gcb '/To Workspace L'],'VariableName',data_L)
  Bus2 : Subsystem  mask{Bus=2}
      mask prompts: Bus "Bus Number"
      mask init:
      | data_V=sprintf('Bus%d',Bus);
      | set_param([gcb '/To Workspace V'],'VariableName',data_V);
      | 
      | data_I=sprintf('I%d',Bus);
      | set_param([gcb '/To Workspace I'],'VariableName',data_I);
  Bus20 : Subsystem  mask{Bus=20}
      mask prompts: Bus "Bus Number"
      mask init:
      | data_V=sprintf('Bus%d',Bus);
      | set_param([gcb '/To Workspace V'],'VariableName',data_V);
      | 
      | data_I=sprintf('I%d',Bus);
      | set_param([gcb '/To Workspace I'],'VariableName',data_I);
  Bus21 : Subsystem  mask{Ph=3, Bus=21, Load=13}
      mask prompts: Ph "Phase [A=1, B=2, C=3]"; Bus "Bus Number"; Load "Load Number"
      mask init:
      | data_V=sprintf('Bus%d',Bus);
      | set_param([gcb '/To Workspace V'],'VariableName',data_V);
      | 
      | data_I=sprintf('I%d',Bus);
      | set_param([gcb '/To Workspace I'],'VariableName',data_I);
      | 
      | data_L=sprintf('Load%d',Load);
      | set_param([gcb '/To Workspace L'],'VariableName',data_L)
  Bus22 : Subsystem  mask{Bus=22}
      mask prompts: Bus "Bus Number"
      mask init:
      | data_V=sprintf('Bus%d',Bus);
      | set_param([gcb '/To Workspace V'],'VariableName',data_V);
      | 
      | data_I=sprintf('I%d',Bus);
      | set_param([gcb '/To Workspace I'],'VariableName',data_I);
  Bus23 : Subsystem  mask{Ph=3, Bus=23, Load=14}
      mask prompts: Ph "Phase [A=1, B=2, C=3]"; Bus "Bus Number"; Load "Load Number"
      mask init:
      | data_V=sprintf('Bus%d',Bus);
      | set_param([gcb '/To Workspace V'],'VariableName',data_V);
      | 
      | data_I=sprintf('I%d',Bus);
      | set_param([gcb '/To Workspace I'],'VariableName',data_I);
      | 
      | data_L=sprintf('Load%d',Load);
      | set_param([gcb '/To Workspace L'],'VariableName',data_L)
  Bus24 : Subsystem  mask{Ph=1, Bus=24, Load=15}
      mask prompts: Ph "Phase [A=1, B=2, C=3]"; Bus "Bus Number"; Load "Load Number"
      mask init:
      | data_V=sprintf('Bus%d',Bus);
      | set_param([gcb '/To Workspace V'],'VariableName',data_V);
      | 
      | data_I=sprintf('I%d',Bus);
      | set_param([gcb '/To Workspace I'],'VariableName',data_I);
      | 
      | data_L=sprintf('Load%d',Load);
      | set_param([gcb '/To Workspace L'],'VariableName',data_L)
  Bus25 : Subsystem  mask{Bus=25}
      mask prompts: Bus "Bus Number"
      mask init:
      | data_V=sprintf('Bus%d',Bus);
      | set_param([gcb '/To Workspace V'],'VariableName',data_V);
      | 
      | data_I=sprintf('I%d',Bus);
      | set_param([gcb '/To Workspace I'],'VariableName',data_I);
  Bus26 : Subsystem  mask{Bus=26, Load=16}
      mask prompts: Bus "Bus Number"; Load "Load Number"
      mask init:
      | data_V=sprintf('Bus%d',Bus);
      | set_param([gcb '/To Workspace V'],'VariableName',data_V);
      | 
      | data_I=sprintf('I%d',Bus);
      | set_param([gcb '/To Workspace I'],'VariableName',data_I);
      | 
      | data_L=sprintf('Load%d',Load);
      | set_param([gcb '/To Workspace L'],'VariableName',data_L)
  Bus27 : Subsystem  mask{Bus=27, Load=17}
      mask prompts: Bus "Bus Number"; Load "Load Number"
      mask init:
      | data_V=sprintf('Bus%d',Bus);
      | set_param([gcb '/To Workspace V'],'VariableName',data_V);
      | 
      | data_I=sprintf('I%d',Bus);
      | set_param([gcb '/To Workspace I'],'VariableName',data_I);
      | 
      | data_L=sprintf('Load%d',Load);
      | set_param([gcb '/To Workspace L'],'VariableName',data_L)
  Bus28 : Subsystem  mask{Ph=3, Bus=28, Load=18}
      mask prompts: Ph "Phase [A=1, B=2, C=3]"; Bus "Bus Number"; Load "Load Number"
      mask init:
      | data_V=sprintf('Bus%d',Bus);
      | set_param([gcb '/To Workspace V'],'VariableName',data_V);
      | 
      | data_I=sprintf('I%d',Bus);
      | set_param([gcb '/To Workspace I'],'VariableName',data_I);
      | 
      | data_L=sprintf('Load%d',Load);
      | set_param([gcb '/To Workspace L'],'VariableName',data_L)
  Bus29 : Subsystem  mask{Ph=2, Bus=29, Load=19}
      mask prompts: Ph "Phase [A=1, B=2, C=3]"; Bus "Bus Number"; Load "Load Number"
      mask init:
      | data_V=sprintf('Bus%d',Bus);
      | set_param([gcb '/To Workspace V'],'VariableName',data_V);
      | 
      | data_I=sprintf('I%d',Bus);
      | set_param([gcb '/To Workspace I'],'VariableName',data_I);
      | 
      | data_L=sprintf('Load%d',Load);
      | set_param([gcb '/To Workspace L'],'VariableName',data_L)
  Bus3 : Subsystem  mask{Bus=3}
      mask prompts: Bus "Bus Number"
      mask init:
      | data_V=sprintf('Bus%d',Bus);
      | set_param([gcb '/To Workspace V'],'VariableName',data_V);
      | 
      | data_I=sprintf('I%d',Bus);
      | set_param([gcb '/To Workspace I'],'VariableName',data_I);
  Bus30 : Subsystem  mask{Bus=30}
      mask prompts: Bus "Bus Number"
      mask init:
      | data_V=sprintf('Bus%d',Bus);
      | set_param([gcb '/To Workspace V'],'VariableName',data_V);
      | 
      | data_I=sprintf('I%d',Bus);
      | set_param([gcb '/To Workspace I'],'VariableName',data_I);
  Bus31 : Subsystem  mask{Bus=31}
      mask prompts: Bus "Bus Number"
      mask init:
      | data_V=sprintf('Bus%d',Bus);
      | set_param([gcb '/To Workspace V'],'VariableName',data_V);
      | 
      | data_I=sprintf('I%d',Bus);
      | set_param([gcb '/To Workspace I'],'VariableName',data_I);
  Bus32 : Subsystem  mask{Ph=2, Bus=32, Load=20}
      mask prompts: Ph "Phase [A=1, B=2, C=3]"; Bus "Bus Number"; Load "Load Number"
      mask init:
      | data_V=sprintf('Bus%d',Bus);
      | set_param([gcb '/To Workspace V'],'VariableName',data_V);
      | 
      | data_I=sprintf('I%d',Bus);
      | set_param([gcb '/To Workspace I'],'VariableName',data_I);
      | 
      | data_L=sprintf('Load%d',Load);
      | set_param([gcb '/To Workspace L'],'VariableName',data_L)
  Bus33 : Subsystem  mask{Bus=33}
      mask prompts: Bus "Bus Number"
      mask init:
      | data_V=sprintf('Bus%d',Bus);
      | set_param([gcb '/To Workspace V'],'VariableName',data_V);
      | 
      | data_I=sprintf('I%d',Bus);
      | set_param([gcb '/To Workspace I'],'VariableName',data_I);
  Bus34 : Subsystem  mask{Ph=2, Bus=34, Load=21}
      mask prompts: Ph "Phase [A=1, B=2, C=3]"; Bus "Bus Number"; Load "Load Number"
      mask init:
      | data_V=sprintf('Bus%d',Bus);
      | set_param([gcb '/To Workspace V'],'VariableName',data_V);
      | 
      | data_I=sprintf('I%d',Bus);
      | set_param([gcb '/To Workspace I'],'VariableName',data_I);
      | 
      | data_L=sprintf('Load%d',Load);
      | set_param([gcb '/To Workspace L'],'VariableName',data_L)
  Bus35 : Subsystem  mask{Ph=1, Bus=35, Load=22}
      mask prompts: Ph "Phase [A=1, B=2, C=3]"; Bus "Bus Number"; Load "Load Number"
      mask init:
      | data_V=sprintf('Bus%d',Bus);
      | set_param([gcb '/To Workspace V'],'VariableName',data_V);
      | 
      | data_I=sprintf('I%d',Bus);
      | set_param([gcb '/To Workspace I'],'VariableName',data_I);
      | 
      | data_L=sprintf('Load%d',Load);
      | set_param([gcb '/To Workspace L'],'VariableName',data_L)
  Bus36 : Subsystem  mask{Ph=3, Bus=36, Load=23}
      mask prompts: Ph "Phase [A=1, B=2, C=3]"; Bus "Bus Number"; Load "Load Number"
      mask init:
      | data_V=sprintf('Bus%d',Bus);
      | set_param([gcb '/To Workspace V'],'VariableName',data_V);
      | 
      | data_I=sprintf('I%d',Bus);
      | set_param([gcb '/To Workspace I'],'VariableName',data_I);
      | 
      | data_L=sprintf('Load%d',Load);
      | set_param([gcb '/To Workspace L'],'VariableName',data_L)
  Bus37 : Subsystem  mask{Ph=1, Bus=37, Load=24}
      mask prompts: Ph "Phase [A=1, B=2, C=3]"; Bus "Bus Number"; Load "Load Number"
      mask init:
      | data_V=sprintf('Bus%d',Bus);
      | set_param([gcb '/To Workspace V'],'VariableName',data_V);
      | 
      | data_I=sprintf('I%d',Bus);
      | set_param([gcb '/To Workspace I'],'VariableName',data_I);
      | 
      | data_L=sprintf('Load%d',Load);
      | set_param([gcb '/To Workspace L'],'VariableName',data_L)
  Bus38 : Subsystem  mask{Ph=3, Bus=38, Load=25}
      mask prompts: Ph "Phase [A=1, B=2, C=3]"; Bus "Bus Number"; Load "Load Number"
      mask init:
      | data_V=sprintf('Bus%d',Bus);
      | set_param([gcb '/To Workspace V'],'VariableName',data_V);
      | 
      | data_I=sprintf('I%d',Bus);
      | set_param([gcb '/To Workspace I'],'VariableName',data_I);
      | 
      | data_L=sprintf('Load%d',Load);
      | set_param([gcb '/To Workspace L'],'VariableName',data_L)
  Bus39 : Subsystem  mask{Bus=39}
      mask prompts: Bus "Bus Number"
      mask init:
      | data_V=sprintf('Bus%d',Bus);
      | set_param([gcb '/To Workspace V'],'VariableName',data_V);
      | 
      | data_I=sprintf('I%d',Bus);
      | set_param([gcb '/To Workspace I'],'VariableName',data_I);
  Bus4 : Subsystem  mask{Bus=4, Load=1}
      mask prompts: Bus "Bus Number"; Load "Load Number"
      mask init:
      | data_V=sprintf('Bus%d',Bus);
      | set_param([gcb '/To Workspace V'],'VariableName',data_V);
      | 
      | data_I=sprintf('I%d',Bus);
      | set_param([gcb '/To Workspace I'],'VariableName',data_I);
      | 
      | data_L=sprintf('Load%d',Load);
      | set_param([gcb '/To Workspace L'],'VariableName',data_L)
  Bus40 : Subsystem  mask{Bus=40, Load=26}
      mask prompts: Bus "Bus Number"; Load "Load Number"
      mask init:
      | data_V=sprintf('Bus%d',Bus);
      | set_param([gcb '/To Workspace V'],'VariableName',data_V);
      | 
      | data_I=sprintf('I%d',Bus);
      | set_param([gcb '/To Workspace I'],'VariableName',data_I);
      | 
      | data_L=sprintf('Load%d',Load);
      | set_param([gcb '/To Workspace L'],'VariableName',data_L)
  Bus41 : Subsystem  mask{Ph=3, Bus=41, Load=27}
      mask prompts: Ph "Phase [A=1, B=2, C=3]"; Bus "Bus Number"; Load "Load Number"
      mask init:
      | data_V=sprintf('Bus%d',Bus);
      | set_param([gcb '/To Workspace V'],'VariableName',data_V);
      | 
      | data_I=sprintf('I%d',Bus);
      | set_param([gcb '/To Workspace I'],'VariableName',data_I);
      | 
      | data_L=sprintf('Load%d',Load);
      | set_param([gcb '/To Workspace L'],'VariableName',data_L)
  Bus42 : Subsystem  mask{Ph=2, Bus=42, Load=28}
      mask prompts: Ph "Phase [A=1, B=2, C=3]"; Bus "Bus Number"; Load "Load Number"
      mask init:
      | data_V=sprintf('Bus%d',Bus);
      | set_param([gcb '/To Workspace V'],'VariableName',data_V);
      | 
      | data_I=sprintf('I%d',Bus);
      | set_param([gcb '/To Workspace I'],'VariableName',data_I);
      | 
      | data_L=sprintf('Load%d',Load);
      | set_param([gcb '/To Workspace L'],'VariableName',data_L)
  Bus43 : Subsystem  mask{Bus=43}
      mask prompts: Bus "Bus Number"
      mask init:
      | data_V=sprintf('Bus%d',Bus);
      | set_param([gcb '/To Workspace V'],'VariableName',data_V);
      | 
      | data_I=sprintf('I%d',Bus);
      | set_param([gcb '/To Workspace I'],'VariableName',data_I);
  Bus44 : Subsystem  mask{Bus=44}
      mask prompts: Bus "Bus Number"
      mask init:
      | data_V=sprintf('Bus%d',Bus);
      | set_param([gcb '/To Workspace V'],'VariableName',data_V);
      | 
      | data_I=sprintf('I%d',Bus);
      | set_param([gcb '/To Workspace I'],'VariableName',data_I);
  Bus45 : Subsystem  mask{Bus=45, Load=29}
      mask prompts: Bus "Bus Number"; Load "Load Number"
      mask init:
      | data_V=sprintf('Bus%d',Bus);
      | set_param([gcb '/To Workspace V'],'VariableName',data_V);
      | 
      | data_I=sprintf('I%d',Bus);
      | set_param([gcb '/To Workspace I'],'VariableName',data_I);
      | 
      | data_L=sprintf('Load%d',Load);
      | set_param([gcb '/To Workspace L'],'VariableName',data_L)
  Bus46 : Subsystem  mask{Bus=46}
      mask prompts: Bus "Bus Number"
      mask init:
      | data_V=sprintf('Bus%d',Bus);
      | set_param([gcb '/To Workspace V'],'VariableName',data_V);
      | 
      | data_I=sprintf('I%d',Bus);
      | set_param([gcb '/To Workspace I'],'VariableName',data_I);
  Bus47 : Subsystem  mask{Ph=3, Bus=47, Load=30}
      mask prompts: Ph "Phase [A=1, B=2, C=3]"; Bus "Bus Number"; Load "Load Number"
      mask init:
      | data_V=sprintf('Bus%d',Bus);
      | set_param([gcb '/To Workspace V'],'VariableName',data_V);
      | 
      | data_I=sprintf('I%d',Bus);
      | set_param([gcb '/To Workspace I'],'VariableName',data_I);
      | 
      | data_L=sprintf('Load%d',Load);
      | set_param([gcb '/To Workspace L'],'VariableName',data_L)
  Bus48 : Subsystem  mask{Ph=2, Bus=48, Load=31}
      mask prompts: Ph "Phase [A=1, B=2, C=3]"; Bus "Bus Number"; Load "Load Number"
      mask init:
      | data_V=sprintf('Bus%d',Bus);
      | set_param([gcb '/To Workspace V'],'VariableName',data_V);
      | 
      | data_I=sprintf('I%d',Bus);
      | set_param([gcb '/To Workspace I'],'VariableName',data_I);
      | 
      | data_L=sprintf('Load%d',Load);
      | set_param([gcb '/To Workspace L'],'VariableName',data_L)
  Bus49 : Subsystem  mask{Bus=49}
      mask prompts: Bus "Bus Number"
      mask init:
      | data_V=sprintf('Bus%d',Bus);
      | set_param([gcb '/To Workspace V'],'VariableName',data_V);
      | 
      | data_I=sprintf('I%d',Bus);
      | set_param([gcb '/To Workspace I'],'VariableName',data_I);
  Bus5 : Subsystem  mask{Bus=5}
      mask prompts: Bus "Bus Number"
      mask init:
      | data_V=sprintf('Bus%d',Bus);
      | set_param([gcb '/To Workspace V'],'VariableName',data_V);
      | 
      | data_I=sprintf('I%d',Bus);
      | set_param([gcb '/To Workspace I'],'VariableName',data_I);
  Bus50 : Subsystem  mask{Bus=50, Load=32}
      mask prompts: Bus "Bus Number"; Load "Load Number"
      mask init:
      | data_V=sprintf('Bus%d',Bus);
      | set_param([gcb '/To Workspace V'],'VariableName',data_V);
      | 
      | data_I=sprintf('I%d',Bus);
      | set_param([gcb '/To Workspace I'],'VariableName',data_I);
      | 
      | data_L=sprintf('Load%d',Load);
      | set_param([gcb '/To Workspace L'],'VariableName',data_L)
  Bus51 : Subsystem  mask{Ph=1, Bus=51, Load=33}
      mask prompts: Ph "Phase [A=1, B=2, C=3]"; Bus "Bus Number"; Load "Load Number"
      mask init:
      | data_V=sprintf('Bus%d',Bus);
      | set_param([gcb '/To Workspace V'],'VariableName',data_V);
      | 
      | data_I=sprintf('I%d',Bus);
      | set_param([gcb '/To Workspace I'],'VariableName',data_I);
      | 
      | data_L=sprintf('Load%d',Load);
      | set_param([gcb '/To Workspace L'],'VariableName',data_L)
  Bus52 : Subsystem  mask{Bus=52}
      mask prompts: Bus "Bus Number"
      mask init:
      | data_V=sprintf('Bus%d',Bus);
      | set_param([gcb '/To Workspace V'],'VariableName',data_V);
      | 
      | data_I=sprintf('I%d',Bus);
      | set_param([gcb '/To Workspace I'],'VariableName',data_I);
  Bus53 : Subsystem  mask{Ph=3, Bus=53, Load=34}
      mask prompts: Ph "Phase [A=1, B=2, C=3]"; Bus "Bus Number"; Load "Load Number"
      mask init:
      | data_V=sprintf('Bus%d',Bus);
      | set_param([gcb '/To Workspace V'],'VariableName',data_V);
      | 
      | data_I=sprintf('I%d',Bus);
      | set_param([gcb '/To Workspace I'],'VariableName',data_I);
      | 
      | data_L=sprintf('Load%d',Load);
      | set_param([gcb '/To Workspace L'],'VariableName',data_L)
  Bus54 : Subsystem  mask{Ph=1, Bus=54, Load=35}
      mask prompts: Ph "Phase [A=1, B=2, C=3]"; Bus "Bus Number"; Load "Load Number"
      mask init:
      | data_V=sprintf('Bus%d',Bus);
      | set_param([gcb '/To Workspace V'],'VariableName',data_V);
      | 
      | data_I=sprintf('I%d',Bus);
      | set_param([gcb '/To Workspace I'],'VariableName',data_I);
      | 
      | data_L=sprintf('Load%d',Load);
      | set_param([gcb '/To Workspace L'],'VariableName',data_L)
  Bus55 : Subsystem  mask{Bus=55}
      mask prompts: Bus "Bus Number"
      mask init:
      | data_V=sprintf('Bus%d',Bus);
      | set_param([gcb '/To Workspace V'],'VariableName',data_V);
      | 
      | data_I=sprintf('I%d',Bus);
      | set_param([gcb '/To Workspace I'],'VariableName',data_I);
  Bus56 : Subsystem  mask{Ph=3, Bus=56, Load=36}
      mask prompts: Ph "Phase [A=1, B=2, C=3]"; Bus "Bus Number"; Load "Load Number"
      mask init:
      | data_V=sprintf('Bus%d',Bus);
      | set_param([gcb '/To Workspace V'],'VariableName',data_V);
      | 
      | data_I=sprintf('I%d',Bus);
      | set_param([gcb '/To Workspace I'],'VariableName',data_I);
      | 
      | data_L=sprintf('Load%d',Load);
      | set_param([gcb '/To Workspace L'],'VariableName',data_L)
  Bus57 : Subsystem  mask{Ph=3, Bus=57, Load=37}
      mask prompts: Ph "Phase [A=1, B=2, C=3]"; Bus "Bus Number"; Load "Load Number"
      mask init:
      | data_V=sprintf('Bus%d',Bus);
      | set_param([gcb '/To Workspace V'],'VariableName',data_V);
      | 
      | data_I=sprintf('I%d',Bus);
      | set_param([gcb '/To Workspace I'],'VariableName',data_I);
      | 
      | data_L=sprintf('Load%d',Load);
      | set_param([gcb '/To Workspace L'],'VariableName',data_L)
  Bus58 : Subsystem  mask{Bus=58}
      mask prompts: Bus "Bus Number"
      mask init:
      | data_V=sprintf('Bus%d',Bus);
      | set_param([gcb '/To Workspace V'],'VariableName',data_V);
      | 
      | data_I=sprintf('I%d',Bus);
      | set_param([gcb '/To Workspace I'],'VariableName',data_I);
  Bus59 : Subsystem  mask{Ph=2, Bus=59, Load=38}
      mask prompts: Ph "Phase [A=1, B=2, C=3]"; Bus "Bus Number"; Load "Load Number"
      mask init:
      | data_V=sprintf('Bus%d',Bus);
      | set_param([gcb '/To Workspace V'],'VariableName',data_V);
      | 
      | data_I=sprintf('I%d',Bus);
      | set_param([gcb '/To Workspace I'],'VariableName',data_I);
      | 
      | data_L=sprintf('Load%d',Load);
      | set_param([gcb '/To Workspace L'],'VariableName',data_L)
  Bus6 : Subsystem  mask{Bus=6, Load=2}
      mask prompts: Bus "Bus Number"; Load "Load Number"
      mask init:
      | data_V=sprintf('Bus%d',Bus);
      | set_param([gcb '/To Workspace V'],'VariableName',data_V);
      | 
      | data_I=sprintf('I%d',Bus);
      | set_param([gcb '/To Workspace I'],'VariableName',data_I);
      | 
      | data_L=sprintf('Load%d',Load);
      | set_param([gcb '/To Workspace L'],'VariableName',data_L)
  Bus60 : Subsystem  mask{Ph=1, Bus=60, Load=39}
      mask prompts: Ph "Phase [A=1, B=2, C=3]"; Bus "Bus Number"; Load "Load Number"
      mask init:
      | data_V=sprintf('Bus%d',Bus);
      | set_param([gcb '/To Workspace V'],'VariableName',data_V);
      | 
      | data_I=sprintf('I%d',Bus);
      | set_param([gcb '/To Workspace I'],'VariableName',data_I);
      | 
      | data_L=sprintf('Load%d',Load);
      | set_param([gcb '/To Workspace L'],'VariableName',data_L)
  Bus61 : Subsystem  mask{Ph=2, Bus=61, Load=40}
      mask prompts: Ph "Phase [A=1, B=2, C=3]"; Bus "Bus Number"; Load "Load Number"
      mask init:
      | data_V=sprintf('Bus%d',Bus);
      | set_param([gcb '/To Workspace V'],'VariableName',data_V);
      | 
      | data_I=sprintf('I%d',Bus);
      | set_param([gcb '/To Workspace I'],'VariableName',data_I);
      | 
      | data_L=sprintf('Load%d',Load);
      | set_param([gcb '/To Workspace L'],'VariableName',data_L)
  Bus62 : Subsystem  mask{Bus=62}
      mask prompts: Bus "Bus Number"
      mask init:
      | data_V=sprintf('Bus%d',Bus);
      | set_param([gcb '/To Workspace V'],'VariableName',data_V);
      | 
      | data_I=sprintf('I%d',Bus);
      | set_param([gcb '/To Workspace I'],'VariableName',data_I);
  Bus63 : Subsystem  mask{Bus=63}
      mask prompts: Bus "Bus Number"
      mask init:
      | data_V=sprintf('Bus%d',Bus);
      | set_param([gcb '/To Workspace V'],'VariableName',data_V);
      | 
      | data_I=sprintf('I%d',Bus);
      | set_param([gcb '/To Workspace I'],'VariableName',data_I);
  Bus64 : Subsystem  mask{Bus=64, Load=41}
      mask prompts: Bus "Bus Number"; Load "Load Number"
      mask init:
      | data_V=sprintf('Bus%d',Bus);
      | set_param([gcb '/To Workspace V'],'VariableName',data_V);
      | 
      | data_I=sprintf('I%d',Bus);
      | set_param([gcb '/To Workspace I'],'VariableName',data_I);
      | 
      | data_L=sprintf('Load%d',Load);
      | set_param([gcb '/To Workspace L'],'VariableName',data_L)
  Bus65 : Subsystem  mask{Ph=3, Bus=65, Load=42}
      mask prompts: Ph "Phase [A=1, B=2, C=3]"; Bus "Bus Number"; Load "Load Number"
      mask init:
      | data_V=sprintf('Bus%d',Bus);
      | set_param([gcb '/To Workspace V'],'VariableName',data_V);
      | 
      | data_I=sprintf('I%d',Bus);
      | set_param([gcb '/To Workspace I'],'VariableName',data_I);
      | 
      | data_L=sprintf('Load%d',Load);
      | set_param([gcb '/To Workspace L'],'VariableName',data_L)
  Bus66 : Subsystem  mask{Bus=66}
      mask prompts: Bus "Bus Number"
      mask init:
      | data_V=sprintf('Bus%d',Bus);
      | set_param([gcb '/To Workspace V'],'VariableName',data_V);
      | 
      | data_I=sprintf('I%d',Bus);
      | set_param([gcb '/To Workspace I'],'VariableName',data_I);
  Bus67 : Subsystem  mask{Ph=1, Bus=67, Load=43}
      mask prompts: Ph "Phase [A=1, B=2, C=3]"; Bus "Bus Number"; Load "Load Number"
      mask init:
      | data_V=sprintf('Bus%d',Bus);
      | set_param([gcb '/To Workspace V'],'VariableName',data_V);
      | 
      | data_I=sprintf('I%d',Bus);
      | set_param([gcb '/To Workspace I'],'VariableName',data_I);
      | 
      | data_L=sprintf('Load%d',Load);
      | set_param([gcb '/To Workspace L'],'VariableName',data_L)
  Bus68 : Subsystem  mask{Ph=3, Bus=68, Load=44}
      mask prompts: Ph "Phase [A=1, B=2, C=3]"; Bus "Bus Number"; Load "Load Number"
      mask init:
      | data_V=sprintf('Bus%d',Bus);
      | set_param([gcb '/To Workspace V'],'VariableName',data_V);
      | 
      | data_I=sprintf('I%d',Bus);
      | set_param([gcb '/To Workspace I'],'VariableName',data_I);
      | 
      | data_L=sprintf('Load%d',Load);
      | set_param([gcb '/To Workspace L'],'VariableName',data_L)
  Bus69 : Subsystem  mask{Ph=2, Bus=69, Load=45}
      mask prompts: Ph "Phase [A=1, B=2, C=3]"; Bus "Bus Number"; Load "Load Number"
      mask init:
      | data_V=sprintf('Bus%d',Bus);
      | set_param([gcb '/To Workspace V'],'VariableName',data_V);
      | 
      | data_I=sprintf('I%d',Bus);
      | set_param([gcb '/To Workspace I'],'VariableName',data_I);
      | 
      | data_L=sprintf('Load%d',Load);
      | set_param([gcb '/To Workspace L'],'VariableName',data_L)
  Bus7 : Subsystem  mask{Ph=1, Bus=7, Load=3}
      mask prompts: Ph "Phase [A=1, B=2, C=3]"; Bus "Bus Number"; Load "Load Number"
      mask init:
      | data_V=sprintf('Bus%d',Bus);
      | set_param([gcb '/To Workspace V'],'VariableName',data_V);
      | 
      | data_I=sprintf('I%d',Bus);
      | set_param([gcb '/To Workspace I'],'VariableName',data_I);
      | 
      | data_L=sprintf('Load%d',Load);
      | set_param([gcb '/To Workspace L'],'VariableName',data_L)
  Bus70 : Subsystem  mask{Bus=70}
      mask prompts: Bus "Bus Number"
      mask init:
      | data_V=sprintf('Bus%d',Bus);
      | set_param([gcb '/To Workspace V'],'VariableName',data_V);
      | 
      | data_I=sprintf('I%d',Bus);
      | set_param([gcb '/To Workspace I'],'VariableName',data_I);
  Bus71 : Subsystem  mask{Ph=1, Bus=71, Load=46}
      mask prompts: Ph "Phase [A=1, B=2, C=3]"; Bus "Bus Number"; Load "Load Number"
      mask init:
      | data_V=sprintf('Bus%d',Bus);
      | set_param([gcb '/To Workspace V'],'VariableName',data_V);
      | 
      | data_I=sprintf('I%d',Bus);
      | set_param([gcb '/To Workspace I'],'VariableName',data_I);
      | 
      | data_L=sprintf('Load%d',Load);
      | set_param([gcb '/To Workspace L'],'VariableName',data_L)
  Bus72 : Subsystem  mask{Ph=2, Bus=72, Load=47}
      mask prompts: Ph "Phase [A=1, B=2, C=3]"; Bus "Bus Number"; Load "Load Number"
      mask init:
      | data_V=sprintf('Bus%d',Bus);
      | set_param([gcb '/To Workspace V'],'VariableName',data_V);
      | 
      | data_I=sprintf('I%d',Bus);
      | set_param([gcb '/To Workspace I'],'VariableName',data_I);
      | 
      | data_L=sprintf('Load%d',Load);
      | set_param([gcb '/To Workspace L'],'VariableName',data_L)
  Bus73 : Subsystem  mask{Ph=3, Bus=73, Load=48}
      mask prompts: Ph "Phase [A=1, B=2, C=3]"; Bus "Bus Number"; Load "Load Number"
      mask init:
      | data_V=sprintf('Bus%d',Bus);
      | set_param([gcb '/To Workspace V'],'VariableName',data_V);
      | 
      | data_I=sprintf('I%d',Bus);
      | set_param([gcb '/To Workspace I'],'VariableName',data_I);
      | 
      | data_L=sprintf('Load%d',Load);
      | set_param([gcb '/To Workspace L'],'VariableName',data_L)
  Bus74 : Subsystem  mask{Bus=74, Load=49}
      mask prompts: Bus "Bus Number"; Load "Load Number"
      mask init:
      | data_V=sprintf('Bus%d',Bus);
      | set_param([gcb '/To Workspace V'],'VariableName',data_V);
      | 
      | data_I=sprintf('I%d',Bus);
      | set_param([gcb '/To Workspace I'],'VariableName',data_I);
      | 
      | data_L=sprintf('Load%d',Load);
      | set_param([gcb '/To Workspace L'],'VariableName',data_L)
  Bus8 : Subsystem  mask{Ph=3, Bus=8, Load=4}
      mask prompts: Ph "Phase [A=1, B=2, C=3]"; Bus "Bus Number"; Load "Load Number"
      mask init:
      | data_V=sprintf('Bus%d',Bus);
      | set_param([gcb '/To Workspace V'],'VariableName',data_V);
      | 
      | data_I=sprintf('I%d',Bus);
      | set_param([gcb '/To Workspace I'],'VariableName',data_I);
      | 
      | data_L=sprintf('Load%d',Load);
      | set_param([gcb '/To Workspace L'],'VariableName',data_L)
  Bus9 : Subsystem  mask{Bus=9}
      mask prompts: Bus "Bus Number"
      mask init:
      | data_V=sprintf('Bus%d',Bus);
      | set_param([gcb '/To Workspace V'],'VariableName',data_V);
      | 
      | data_I=sprintf('I%d',Bus);
      | set_param([gcb '/To Workspace I'],'VariableName',data_I);
  Ground1 : powerlib/Elements/Ground  LConnTagsString=a
  Load1 : Subsystem
  Load10 : Subsystem
  Load11 : Subsystem
  Load12 : Subsystem
  Load13 : Subsystem
  Load14 : Subsystem
  Load15 : Subsystem
  Load16 : Subsystem
  Load17 : Subsystem
  Load18 : Subsystem
  Load19 : Subsystem
  Load2 : Subsystem
  Load20 : Subsystem
  Load21 : Subsystem
  Load22 : Subsystem
  Load23 : Subsystem
  Load24 : Subsystem
  Load25 : Subsystem
  Load26 : Subsystem
  Load27 : Subsystem
  Load28 : Subsystem
  Load29 : Subsystem
  Load3 : Subsystem
  Load30 : Subsystem
  Load31 : Subsystem
  Load32 : Subsystem
  Load33 : Subsystem
  Load34 : Subsystem
  Load35 : Subsystem
  Load36 : Subsystem
  Load37 : Subsystem
  Load38 : Subsystem
  Load39 : Subsystem
  Load4 : Subsystem
  Load40 : Subsystem
  Load41 : Subsystem
  Load42 : Subsystem
  Load43 : Subsystem
  Load44 : Subsystem
  Load45 : Subsystem
  Load46 : Subsystem
  Load47 : Subsystem
  Load48 : Subsystem
  Load49 : Subsystem
  Load5 : Subsystem
  Load6 : Subsystem
  Load7 : Subsystem
  Load8 : Subsystem
  Load9 : Subsystem
  SS : Subsystem  mask{MV_grid=Source_Voltage, OLTC=off, Vtarget=1.025, Tap_Value=0.0125, tap_num=8, deadband=0.015}
      mask prompts: MV_grid "Source voltage for MV grid"; OLTC "Enable OLTC"; Vtarget "Target Voltage [pu]"; Tap_Value "Tap Value [pu]"; tap_num "Number of tap positions"; deadband "Tap deadband [pu]"
      mask init:
      | % OLTC = get_param(gcb,'OLTC');
      | % block_OLTC=find_system(gcb,'LookUnderMasks','on','IncludeCommented','on','Name','OLTC');
      | % block_Normal=find_system(gcb,'LookUnderMasks','on','IncludeCommented','on','Name','Normal');
      | % 
      | % if strcmp(OLTC,'off')
      | %     set_param(char(block_OLTC),'Commented','on');
      | %     set_param(char(block_Normal),'Commented','off');
      | % else
      | %     set_param(char(block_OLTC),'Commented','off');
      | %     set_param(char(block_Normal),'Commented','on');
      | % end
  XLPE 185/90 Line 1 : myLibrary/4-Wire Cable  R=R_xlpe_185_90  L=L_xlpe_185_90  C=C_xlpe_185_90  Length=Line_length(2)
  XLPE 185/90 Line 2 : myLibrary/4-Wire Cable  R=R_xlpe_185_90  L=L_xlpe_185_90  C=C_xlpe_185_90  Length=Line_length(3)
  XLPE 185/90 Line 3 : myLibrary/4-Wire Cable  R=R_xlpe_185_90  L=L_xlpe_185_90  C=C_xlpe_185_90  Length=Line_length(4)
  powergui : powerlib/powergui  Priority=1  SimulationMode=Phasor  SampleTime=900  frequency=50  Iterations=50  frequencyindice=50  Pbase=100e6  ErrMax=1e-4  UnitsV=kV  UnitsW=MW  buscounter=0  FunctionMessages=off  echomessages=off  EnableUseOfTLC=off  CurrentSourceSwitches=off  DisableSnubberDevices=off  DisableRonSwitches=off  DisableVfSwitches=off  DisplayEquations=off  AutomaticDiscreteSolvers=off  SolverType=Tustin/Backward Euler (TBE)  Interpol=off  ExternalGateDelay=off  methode=off  Ts=100  x0status=blocks  SPID=off  SwTol=0  HookPort=off  NonlinearTolerance=1e-4  nMaxIteration=100  ContinueOnMaxIteration=off  RestoreLinks=warning  ResistiveCurrentMeasurement=off  Frange=[0:2:500]  Ylog=off  Xlog=on  ShowGrid=off  save=off  variable=ZData  structure=0  ZoomFFT=off  StartTime=0.0  cycles=1  DisplayStyle=1  fundamental=60  FreqAxis=off  MaxFrequency=1000  frequencyindicesteady=1  RmsSteady=1  display=off
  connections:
  Bus2/LConn4 -- Ground1/LConn1
  Bus1/LConn2 -- SS/RConn2
  Bus1/LConn1 -- SS/RConn1
  Bus1/LConn3 -- SS/RConn3
  Bus1/LConn4 -- SS/RConn4
  Bus46/RConn2 -- 22mm^2 Line 46/RConn1 -- 100mm^2 Line 47/RConn2
  100mm^2 Line 23/LConn3 -- 22mm^2 Line 21/RConn1 -- Bus22/RConn3
  50mm^2 Line 56/RConn4 -- 22mm^2 Line 54/RConn2 -- 22mm^2 Line 55/RConn2 -- Bus55/RConn4
  Bus20/RConn4 -- 22mm^2 Line 19/RConn2 -- 100mm^2 Line 20/LConn4
  22mm^2 Line 33/RConn2 -- Bus33/RConn4 -- 22mm^2 Line 32/LConn2
  Bus39/RConn3 -- 22mm^2 Line 38/LConn3 -- 100mm^2 Line 41/RConn3 -- 22mm^2 Line 39/RConn1
  22mm^2 Line 40/RConn2 -- 22mm^2 Line 38/LConn4 -- Bus39/RConn4 -- 22mm^2 Line 39/RConn2 -- 100mm^2 Line 41/RConn4
  Bus62/RConn2 -- 22mm^2 Line 67/RConn1 -- 50mm^2 Line 61/RConn2 -- 100mm^2 Line 68/LConn2
  22mm^2 Line 11/RConn2 -- 16mm^2 Line 8/LConn2 -- Bus9/RConn4 -- 22mm^2 Line 10/RConn2 -- 100mm^2 Line 12/LConn4 -- 22mm^2 Line 9/LConn2
  100mm^2 Line 50/RConn3 -- 22mm^2 Line 48/LConn3 -- Bus49/RConn3
  22mm^2 Line 72/LConn3 -- 22mm^2 Line 71/RConn1 -- Bus70/RConn3
  Bus58/RConn4 -- 22mm^2 Line 57/RConn2 -- 50mm^2 Line 60/RConn4 -- 22mm^2 Line 58/RConn2 -- 22mm^2 Line 59/RConn2
  Bus16/RConn4 -- 22mm^2 Line 15/RConn2 -- 100mm^2 Line 28/LConn4 -- 100mm^2 Line 18/LConn4 -- 22mm^2 Line 16/RConn2 -- 22mm^2 Line 17/LConn2
  100mm^2 Line 29/LConn4 -- 100mm^2 Line 37/RConn4 -- Bus30/RConn4 -- 22mm^2 Line 36/RConn2 -- 16mm^2 Line 34/LConn2 -- 22mm^2 Line 35/LConn2
  16mm^2 Line 24/LConn3 -- Bus25/RConn3 -- 22mm^2 Line 26/LConn1 -- 16mm^2 Line 25/LConn3
  50mm^2 Line 60/RConn3 -- Bus58/RConn3
  16mm^2 Line 24/LConn2 -- 16mm^2 Line 25/LConn2 -- Bus25/RConn2 -- 22mm^2 Line 27/LConn1
  Bus30/RConn1 -- 100mm^2 Line 29/LConn1 -- 22mm^2 Line 35/LConn1 -- 100mm^2 Line 37/RConn1
  100mm^2 Line 28/LConn1 -- 100mm^2 Line 18/LConn1 -- Bus16/RConn1
  Bus30/RConn3 -- 100mm^2 Line 29/LConn3 -- 100mm^2 Line 37/RConn3 -- 22mm^2 Line 36/RConn1 -- 16mm^2 Line 34/LConn1
  Bus22/RConn4 -- 22mm^2 Line 21/RConn2 -- 100mm^2 Line 23/LConn4 -- 22mm^2 Line 22/RConn2
  100mm^2 Line 20/LConn3 -- 22mm^2 Line 19/RConn1 -- Bus20/RConn3
  50mm^2 Line 64/RConn1 -- 16mm^2 Line 62/LConn1 -- Bus63/RConn1
  Bus49/RConn2 -- 22mm^2 Line 48/LConn2 -- 100mm^2 Line 50/RConn2
  Bus39/RConn1 -- 22mm^2 Line 38/LConn1 -- 100mm^2 Line 41/RConn1
  Bus22/RConn1 -- 22mm^2 Line 22/RConn1 -- 100mm^2 Line 23/LConn1
  100mm^2 Line 44/RConn1 -- 100mm^2 Line 42/RConn1 -- Bus43/RConn1
  22mm^2 Line 13/LConn1 -- Bus14/RConn1 -- 100mm^2 Line 14/LConn1
  Bus9/RConn1 -- 22mm^2 Line 11/RConn1 -- 100mm^2 Line 12/LConn1
  Bus43/RConn4 -- 100mm^2 Line 42/RConn4 -- 100mm^2 Line 44/RConn4
  50mm^2 Line 53/RConn1 -- 22mm^2 Line 52/LConn1 -- Bus52/RConn1
  22mm^2 Line 6/RConn2 -- Bus5/RConn4 -- 22mm^2 Line 4/LConn4 -- 100mm^2 Line 7/LConn4 -- 22mm^2 Line 5/LConn2
  XLPE 185/90 Line 2/LConn2 -- Bus3/RConn2 -- XLPE 185/90 Line 3/LConn2
  Bus46/RConn3 -- 22mm^2 Line 45/LConn1 -- 100mm^2 Line 47/RConn3
  22mm^2 Line 66/RConn2 -- 50mm^2 Line 61/RConn4 -- 100mm^2 Line 68/LConn4 -- Bus62/RConn4 -- 22mm^2 Line 65/RConn2 -- 22mm^2 Line 67/RConn2
  22mm^2 Line 4/LConn3 -- Bus5/RConn3 -- 100mm^2 Line 7/LConn3 -- 22mm^2 Line 6/RConn1
  22mm^2 Line 72/LConn4 -- 22mm^2 Line 71/RConn2 -- Bus70/RConn4 -- 22mm^2 Line 69/RConn2 -- 22mm^2 Line 70/RConn2
  16mm^2 Line 62/LConn4 -- Bus63/RConn4 -- 50mm^2 Line 64/RConn4 -- 22mm^2 Line 63/RConn2
  16mm^2 Line 24/LConn1 -- Bus25/RConn1 -- 16mm^2 Line 25/LConn1
  100mm^2 Line 18/LConn3 -- 22mm^2 Line 15/RConn1 -- 22mm^2 Line 17/LConn1 -- Bus16/RConn3 -- 22mm^2 Line 16/RConn1 -- 100mm^2 Line 28/LConn3
  22mm^2 Line 13/LConn2 -- Bus14/RConn4 -- 100mm^2 Line 14/LConn4
  50mm^2 Line 60/RConn1 -- 22mm^2 Line 58/RConn1 -- Bus58/RConn1
  Bus43/RConn3 -- 100mm^2 Line 42/RConn3 -- 100mm^2 Line 44/RConn3
  22mm^2 Line 40/RConn1 -- 22mm^2 Line 38/LConn2 -- Bus39/RConn2 -- 100mm^2 Line 41/RConn2
  100mm^2 Line 50/RConn1 -- 22mm^2 Line 48/LConn1 -- 22mm^2 Line 49/RConn1 -- Bus49/RConn1
  Load10/LConn2 -- Bus17/RConn2
  16mm^2 Line 24/LConn4 -- 16mm^2 Line 25/LConn4 -- Bus25/RConn4 -- 22mm^2 Line 27/LConn2 -- 22mm^2 Line 26/LConn2
  22mm^2 Line 59/RConn1 -- 50mm^2 Line 60/RConn2 -- 22mm^2 Line 57/RConn1 -- Bus58/RConn2
  22mm^2 Line 4/LConn2 -- Bus5/RConn2 -- 100mm^2 Line 7/LConn2
  Load28/LConn2 -- Bus42/RConn2
  22mm^2 Line 5/LConn1 -- 22mm^2 Line 4/LConn1 -- Bus5/RConn1 -- 100mm^2 Line 7/LConn1
  22mm^2 Line 69/RConn1 -- Bus70/RConn1 -- 22mm^2 Line 72/LConn1
  Bus46/RConn4 -- 22mm^2 Line 46/RConn2 -- 100mm^2 Line 47/RConn4 -- 22mm^2 Line 45/LConn2
  100mm^2 Line 44/RConn2 -- 100mm^2 Line 42/RConn2 -- Bus43/RConn2
  22mm^2 Line 66/RConn1 -- 50mm^2 Line 61/RConn3 -- 100mm^2 Line 68/LConn3 -- Bus62/RConn3
  22mm^2 Line 49/RConn2 -- 22mm^2 Line 48/LConn4 -- Bus49/RConn4 -- 100mm^2 Line 50/RConn4
  100mm^2 Line 28/LConn2 -- 100mm^2 Line 18/LConn2 -- Bus16/RConn2
  50mm^2 Line 56/RConn3 -- 22mm^2 Line 54/RConn1 -- 22mm^2 Line 55/RConn1 -- Bus55/RConn3
  Bus52/RConn3 -- 22mm^2 Line 51/RConn1 -- 50mm^2 Line 53/RConn3
  Bus63/RConn3 -- 16mm^2 Line 62/LConn3 -- 50mm^2 Line 64/RConn3 -- 22mm^2 Line 63/RConn1
  XLPE 185/90 Line 2/LConn3 -- Bus3/RConn3 -- XLPE 185/90 Line 3/LConn3
  50mm^2 Line 61/RConn1 -- 100mm^2 Line 68/LConn1 -- 22mm^2 Line 65/RConn1 -- Bus62/RConn1
  22mm^2 Line 30/LConn1 -- Bus31/RConn2 -- 100mm^2 Line 31/LConn2
  Bus7/RConn2 -- Load3/LConn2
  Load3/LConn1 -- Bus7/RConn1
  22mm^2 Line 30/LConn2 -- Bus31/RConn4 -- 100mm^2 Line 31/LConn4
  22mm^2 Line 10/RConn1 -- 22mm^2 Line 9/LConn1 -- 100mm^2 Line 12/LConn2 -- Bus9/RConn2
  XLPE 185/90 Line 2/LConn1 -- Bus3/RConn1 -- XLPE 185/90 Line 3/LConn1
  100mm^2 Line 29/LConn2 -- Bus30/RConn2 -- 100mm^2 Line 37/RConn2
  Load10/LConn1 -- Bus17/RConn1
  100mm^2 Line 12/LConn3 -- 16mm^2 Line 8/LConn1 -- Bus9/RConn3
  Bus52/RConn4 -- 22mm^2 Line 52/LConn2 -- 50mm^2 Line 53/RConn4 -- 22mm^2 Line 51/RConn2
  16mm^2 Line 62/LConn2 -- Bus63/RConn2 -- 50mm^2 Line 64/RConn2
  Load28/LConn1 -- Bus42/RConn1
  22mm^2 Line 70/RConn1 -- Bus70/RConn2 -- 22mm^2 Line 72/LConn2
  XLPE 185/90 Line 2/LConn4 -- Bus3/RConn4 -- XLPE 185/90 Line 3/LConn4
  16mm^2 Line 62/RConn3 -- Bus64/LConn3
  Bus36/RConn2 -- Load23/LConn2
  Bus65/RConn2 -- Load42/LConn2
  Bus62/LConn3 -- 50mm^2 Line 60/LConn3
  100mm^2 Line 14/LConn3 -- Bus14/RConn3
  Bus50/RConn4 -- Load32/LConn4
  100mm^2 Line 28/RConn1 -- Bus30/LConn1
  Load4/LConn1 -- Bus8/RConn1
  22mm^2 Line 5/RConn2 -- Bus7/LConn2
  Bus38/RConn1 -- Load25/LConn1
  50mm^2 Line 56/RConn2 -- Bus55/RConn2
  Bus61/RConn2 -- Load40/LConn2
  Bus68/RConn1 -- Load44/LConn1
  22mm^2 Line 9/RConn2 -- Bus11/LConn2
  Bus59/RConn1 -- Load38/LConn1
  Bus61/LConn2 -- 22mm^2 Line 59/LConn2
  16mm^2 Line 62/RConn1 -- Bus64/LConn1
  Bus22/LConn2 -- 100mm^2 Line 20/RConn2
  22mm^2 Line 71/LConn1 -- Bus73/LConn1
  Bus9/LConn1 -- 100mm^2 Line 7/RConn1
  XLPE 185/90 Line 1/RConn2 -- Bus3/LConn2
  Bus67/LConn2 -- 22mm^2 Line 65/LConn2
  Bus59/RConn2 -- Load38/LConn2
  Bus36/LConn2 -- 16mm^2 Line 34/RConn2
  Bus40/LConn1 -- 22mm^2 Line 38/RConn1
  Bus69/RConn2 -- Load45/LConn2
  Bus13/LConn2 -- 22mm^2 Line 11/LConn2
  Bus69/LConn2 -- 22mm^2 Line 67/LConn2
  Bus57/LConn1 -- 22mm^2 Line 55/LConn1
  Load5/LConn1 -- Bus10/RConn1
  Bus49/LConn2 -- 100mm^2 Line 47/LConn2
  100mm^2 Line 20/LConn2 -- Bus20/RConn2
  Bus48/LConn1 -- 22mm^2 Line 46/LConn1
  Bus55/LConn4 -- 50mm^2 Line 53/LConn4
  Bus60/RConn2 -- Load39/LConn2
  Bus26/RConn2 -- Load16/LConn2
  Bus68/LConn1 -- 22mm^2 Line 66/LConn1
  Bus66/LConn2 -- 50mm^2 Line 64/LConn2
  Bus61/RConn1 -- Load40/LConn1
  Bus60/RConn1 -- Load39/LConn1
  100mm^2 Line 47/RConn1 -- Bus46/RConn1
  Bus68/RConn2 -- Load44/LConn2
  22mm^2 Line 58/LConn1 -- Bus60/LConn1
  Bus23/RConn2 -- Load14/LConn2
  Bus63/LConn4 -- 50mm^2 Line 61/LConn4
  Bus57/LConn2 -- 22mm^2 Line 55/LConn2
  Bus34/LConn2 -- 22mm^2 Line 32/RConn2
  Load21/LConn1 -- Bus34/RConn1
  Bus37/LConn1 -- 22mm^2 Line 35/RConn1
  Bus18/LConn2 -- 22mm^2 Line 16/LConn2
  Bus50/RConn3 -- Load32/LConn3
  22mm^2 Line 43/LConn1 -- Bus44/RConn1
  Bus56/RConn2 -- Load36/LConn2
  Bus58/LConn3 -- 50mm^2 Line 56/LConn3
  22mm^2 Line 9/RConn1 -- Bus11/LConn1
  Bus56/LConn1 -- 22mm^2 Line 54/LConn1
  Bus9/LConn4 -- 100mm^2 Line 7/RConn4
  22mm^2 Line 57/LConn1 -- Bus59/LConn1
  Bus60/LConn2 -- 22mm^2 Line 58/LConn2
  100mm^2 Line 31/LConn1 -- Bus31/RConn1
  Bus33/LConn3 -- 100mm^2 Line 31/RConn3
  Bus38/LConn2 -- 22mm^2 Line 36/LConn2
  Bus22/LConn1 -- 100mm^2 Line 20/RConn1
  22mm^2 Line 72/RConn1 -- Bus74/LConn1
  16mm^2 Line 24/RConn1 -- Bus26/LConn1
  Bus23/LConn2 -- 22mm^2 Line 21/LConn2
  Load9/LConn2 -- Bus15/RConn2
  Bus57/RConn2 -- Load37/LConn2
  Bus26/LConn4 -- 16mm^2 Line 24/RConn4
  Bus74/RConn1 -- Load49/LConn1
  Bus45/RConn3 -- Load29/LConn3
  Bus33/RConn2 -- 22mm^2 Line 32/LConn1
  Bus4/LConn1 -- XLPE 185/90 Line 2/RConn1
  Bus39/LConn1 -- 100mm^2 Line 37/LConn1
  Bus37/LConn2 -- 22mm^2 Line 35/RConn2
  Bus19/RConn2 -- Load12/LConn2
  Bus58/LConn1 -- 50mm^2 Line 56/LConn1
  Load26/LConn3 -- Bus40/RConn3
  Bus49/LConn1 -- 100mm^2 Line 47/LConn1
  Bus56/RConn1 -- Load36/LConn1
  Load7/LConn1 -- Bus12/RConn1
  Load1/LConn4 -- Bus4/RConn4
  Bus43/LConn4 -- 100mm^2 Line 41/LConn4
  Bus67/RConn1 -- Load43/LConn1
  Load1/LConn1 -- Bus4/RConn1
  Bus22/LConn3 -- 100mm^2 Line 20/RConn3
  Bus20/LConn4 -- 100mm^2 Line 18/RConn4
  Bus24/LConn2 -- 22mm^2 Line 22/LConn2
  Bus53/LConn2 -- 22mm^2 Line 51/LConn2
  Bus18/LConn1 -- 22mm^2 Line 16/LConn1
  Bus50/LConn3 -- 22mm^2 Line 48/RConn3
  Bus54/LConn2 -- 22mm^2 Line 52/RConn2
  Bus48/LConn2 -- 22mm^2 Line 46/LConn2
  Bus67/RConn2 -- Load43/LConn2
  Bus65/LConn2 -- 22mm^2 Line 63/LConn2
  Bus42/LConn1 -- 22mm^2 Line 40/LConn1
  Load26/LConn1 -- Bus40/RConn1
  Bus72/RConn1 -- Load47/LConn1
  Bus47/LConn1 -- 22mm^2 Line 45/RConn1
  Bus6/LConn4 -- 22mm^2 Line 4/RConn4
  Load18/LConn2 -- Bus28/RConn2
  Bus66/LConn4 -- 50mm^2 Line 64/LConn4
  Bus51/LConn2 -- 22mm^2 Line 49/LConn2
  Bus23/LConn1 -- 22mm^2 Line 21/LConn1
  Bus32/LConn2 -- 22mm^2 Line 30/RConn2
  Bus47/RConn2 -- Load30/LConn2
  Bus45/RConn4 -- Load29/LConn4
  XLPE 185/90 Line 1/RConn1 -- Bus3/LConn1
  100mm^2 Line 31/LConn3 -- Bus31/RConn3
  Bus66/LConn1 -- 50mm^2 Line 64/LConn1
  Bus41/LConn1 -- 22mm^2 Line 39/LConn1
  Load1/LConn3 -- Bus4/RConn3
  Load6/LConn1 -- Bus11/RConn1
  Bus20/LConn1 -- 100mm^2 Line 18/RConn1
  22mm^2 Line 43/LConn2 -- Bus44/RConn2
  Bus44/LConn4 -- 100mm^2 Line 42/LConn4
  Bus73/LConn2 -- 22mm^2 Line 71/LConn2
  Bus6/RConn3 -- Load2/LConn3
  Bus63/LConn3 -- 50mm^2 Line 61/LConn3
  100mm^2 Line 28/RConn4 -- Bus30/LConn4
  Bus31/LConn3 -- 100mm^2 Line 29/RConn3
  Bus27/RConn1 -- Load17/LConn1
  Load7/LConn2 -- Bus12/RConn2
  Bus16/LConn1 -- 100mm^2 Line 14/RConn1
  Bus26/RConn1 -- Load16/LConn1
  Bus4/LConn3 -- XLPE 185/90 Line 2/RConn3
  Bus58/LConn2 -- 50mm^2 Line 56/LConn2
  Bus71/LConn2 -- 22mm^2 Line 69/LConn2
  22mm^2 Line 33/RConn1 -- Bus33/RConn1
  Bus37/RConn2 -- Load24/LConn2
  Load26/LConn2 -- Bus40/RConn2
  Bus46/LConn4 -- 100mm^2 Line 44/LConn4
  22mm^2 Line 72/RConn3 -- Bus74/LConn3
  Bus49/LConn4 -- 100mm^2 Line 47/LConn4
  Bus38/LConn1 -- 22mm^2 Line 36/LConn1
  Bus2/RConn3 -- XLPE 185/90 Line 1/LConn3
  Bus33/LConn2 -- 100mm^2 Line 31/RConn2
  16mm^2 Line 25/RConn2 -- Bus27/LConn2
  22mm^2 Line 43/LConn4 -- Bus44/RConn4
  Bus50/LConn1 -- 22mm^2 Line 48/RConn1
  XLPE 185/90 Line 1/RConn4 -- Bus3/LConn4
  Bus72/LConn2 -- 22mm^2 Line 70/LConn2
  Bus25/LConn1 -- 100mm^2 Line 23/RConn1
  Bus17/LConn2 -- 22mm^2 Line 15/LConn2
  Load18/LConn1 -- Bus28/RConn1
  Bus25/LConn4 -- 100mm^2 Line 23/RConn4
  Bus26/LConn2 -- 16mm^2 Line 24/RConn2
  Bus24/RConn2 -- Load15/LConn2
  Bus19/LConn1 -- 22mm^2 Line 17/RConn1
  Bus56/LConn2 -- 22mm^2 Line 54/LConn2
  Load4/LConn2 -- Bus8/RConn2
  Load27/LConn2 -- Bus41/RConn2
  Bus31/LConn1 -- 100mm^2 Line 29/RConn1
  Bus8/LConn2 -- 22mm^2 Line 6/LConn2
  Load5/LConn2 -- Bus10/RConn2
  Bus24/LConn1 -- 22mm^2 Line 22/LConn1
  16mm^2 Line 24/RConn3 -- Bus26/LConn3
  100mm^2 Line 23/LConn2 -- Bus22/RConn2
  Bus31/LConn2 -- 100mm^2 Line 29/RConn2
  Bus27/RConn2 -- Load17/LConn2
  Bus73/RConn1 -- Load48/LConn1
  Bus45/LConn2 -- 22mm^2 Line 43/RConn2
  Bus25/LConn3 -- 100mm^2 Line 23/RConn3
  16mm^2 Line 25/RConn1 -- Bus27/LConn1
  Bus47/LConn2 -- 22mm^2 Line 45/RConn2
  Bus35/LConn1 -- 22mm^2 Line 33/LConn1
  Bus27/RConn4 -- Load17/LConn4
  Bus23/RConn1 -- Load14/LConn1
  Bus26/RConn4 -- Load16/LConn4
  Bus21/LConn2 -- 22mm^2 Line 19/LConn2
  Bus64/LConn4 -- 16mm^2 Line 62/RConn4
  Bus24/RConn1 -- Load15/LConn1
  22mm^2 Line 13/RConn2 -- Bus15/LConn2
  Load19/LConn1 -- Bus29/RConn1
  Bus73/RConn2 -- Load48/LConn2
  Bus22/LConn4 -- 100mm^2 Line 20/RConn4
  Bus54/LConn1 -- 22mm^2 Line 52/RConn1
  Bus51/RConn2 -- Load33/LConn2
  Bus16/LConn2 -- 100mm^2 Line 14/RConn2
  Bus64/RConn3 -- Load41/LConn3
  Bus21/RConn1 -- Load13/LConn1
  Bus54/RConn2 -- Load35/LConn2
  Bus12/LConn2 -- 22mm^2 Line 10/LConn2
  Bus70/LConn4 -- 100mm^2 Line 68/RConn4
  Bus12/LConn1 -- 22mm^2 Line 10/LConn1
  Bus14/LConn1 -- 100mm^2 Line 12/RConn1
  Bus38/RConn2 -- Load25/LConn2
  Bus40/LConn2 -- 22mm^2 Line 38/RConn2
  Bus6/RConn1 -- Load2/LConn1
  Bus54/RConn1 -- Load35/LConn1
  Load12/LConn1 -- Bus19/RConn1
  Bus14/LConn2 -- 100mm^2 Line 12/RConn2
  Bus45/RConn1 -- Load29/LConn1
  50mm^2 Line 53/RConn2 -- Bus52/RConn2
  22mm^2 Line 13/RConn1 -- Bus15/LConn1
  Bus18/RConn2 -- Load11/LConn2
  Bus5/LConn1 -- XLPE 185/90 Line 3/RConn1
  Bus16/LConn4 -- 100mm^2 Line 14/RConn4
  Bus64/RConn1 -- Load41/LConn1
  Bus6/RConn4 -- Load2/LConn4
  Bus55/LConn3 -- 50mm^2 Line 53/LConn3
  22mm^2 Line 4/RConn1 -- Bus6/LConn1
  Bus9/LConn3 -- 100mm^2 Line 7/RConn3
  Bus35/RConn2 -- Load22/LConn2
  Bus6/LConn2 -- 22mm^2 Line 4/RConn2
  Bus70/LConn1 -- 100mm^2 Line 68/RConn1
  Load24/LConn1 -- Bus37/RConn1
  22mm^2 Line 67/LConn1 -- Bus69/LConn1
  Bus69/RConn1 -- Load45/LConn1
  Load6/LConn2 -- Bus11/RConn2
  16mm^2 Line 25/RConn3 -- Bus27/LConn3
  22mm^2 Line 27/RConn2 -- Bus29/LConn2
  Bus21/RConn2 -- Load13/LConn2
  Bus58/LConn4 -- 50mm^2 Line 56/LConn4
  Bus10/LConn1 -- 16mm^2 Line 8/RConn1
  Bus63/LConn1 -- 50mm^2 Line 61/LConn1
  Bus2/RConn2 -- XLPE 185/90 Line 1/LConn2
  Bus65/LConn1 -- 22mm^2 Line 63/LConn1
  22mm^2 Line 26/RConn2 -- Bus28/LConn2
  Bus2/RConn4 -- XLPE 185/90 Line 1/LConn4
  Bus34/RConn2 -- Load21/LConn2
  Bus66/LConn3 -- 50mm^2 Line 64/LConn3
  Bus70/LConn3 -- 100mm^2 Line 68/RConn3
  Bus59/LConn2 -- 22mm^2 Line 57/LConn2
  Bus4/LConn4 -- XLPE 185/90 Line 2/RConn4
  Bus74/RConn3 -- Load49/LConn3
  Bus74/RConn2 -- Load49/LConn2
  Bus42/LConn2 -- 22mm^2 Line 40/LConn2
  Bus45/LConn4 -- 22mm^2 Line 43/RConn4
  Bus14/LConn4 -- 100mm^2 Line 12/RConn4
  Bus13/LConn1 -- 22mm^2 Line 11/LConn1
  Bus52/LConn1 -- 100mm^2 Line 50/LConn1
  Bus50/LConn2 -- 22mm^2 Line 48/RConn2
  22mm^2 Line 43/LConn3 -- Bus44/RConn3
  Bus50/RConn1 -- Load32/LConn1
  Bus39/LConn2 -- 100mm^2 Line 37/LConn2
  Bus33/LConn4 -- 100mm^2 Line 31/RConn4
  22mm^2 Line 4/RConn3 -- Bus6/LConn3
  Bus74/LConn4 -- 22mm^2 Line 72/RConn4
  Bus72/RConn2 -- Load47/LConn2
  Load23/LConn1 -- Bus36/RConn1
  Load8/LConn2 -- Bus13/RConn2
  Bus52/LConn3 -- 100mm^2 Line 50/LConn3
  22mm^2 Line 26/RConn1 -- Bus28/LConn1
  Bus43/LConn1 -- 100mm^2 Line 41/LConn1
  Bus63/LConn2 -- 50mm^2 Line 61/LConn2
  Bus67/LConn1 -- 22mm^2 Line 65/LConn1
  Load9/LConn1 -- Bus15/RConn1
  Bus52/LConn2 -- 100mm^2 Line 50/LConn2
  Bus35/RConn1 -- Load22/LConn1
  Bus26/RConn3 -- Load16/LConn3
  Bus45/RConn2 -- Load29/LConn2
  100mm^2 Line 37/LConn4 -- Bus39/LConn4
  Bus57/RConn1 -- Load37/LConn1
  Bus34/LConn1 -- 22mm^2 Line 32/RConn1
  Bus32/LConn1 -- 22mm^2 Line 30/RConn1
  50mm^2 Line 56/RConn1 -- Bus55/RConn1
  Load8/LConn1 -- Bus13/RConn1
  Bus33/LConn1 -- 100mm^2 Line 31/RConn1
  Bus68/LConn2 -- 22mm^2 Line 66/LConn2
  Bus40/LConn3 -- 22mm^2 Line 38/RConn3
  Bus16/LConn3 -- 100mm^2 Line 14/RConn3
  Bus35/LConn2 -- 22mm^2 Line 33/LConn2
  Bus21/LConn1 -- 22mm^2 Line 19/LConn1
  22mm^2 Line 69/LConn1 -- Bus71/LConn1
  XLPE 185/90 Line 1/RConn3 -- Bus3/LConn3
  Bus5/LConn2 -- XLPE 185/90 Line 3/RConn2
  Load1/LConn2 -- Bus4/RConn2
  Bus27/RConn3 -- Load17/LConn3
  Bus40/LConn4 -- 22mm^2 Line 38/RConn4
  Bus71/RConn2 -- Load46/LConn2
  Bus51/RConn1 -- Load33/LConn1
  Bus49/LConn3 -- 100mm^2 Line 47/LConn3
  Bus61/LConn1 -- 22mm^2 Line 59/LConn1
  16mm^2 Line 25/RConn4 -- Bus27/LConn4
  Bus50/RConn2 -- Load32/LConn2
  Bus48/RConn1 -- Load31/LConn1
  Bus4/LConn2 -- XLPE 185/90 Line 2/RConn2
  Bus64/RConn4 -- Load41/LConn4
  Bus55/LConn2 -- 50mm^2 Line 53/LConn2
  Bus62/LConn4 -- 50mm^2 Line 60/LConn4
  Bus5/LConn4 -- XLPE 185/90 Line 3/RConn4
  Bus48/RConn2 -- Load31/LConn2
  Bus64/LConn2 -- 16mm^2 Line 62/RConn2
  Bus51/LConn1 -- 22mm^2 Line 49/LConn1
  Bus45/LConn1 -- 22mm^2 Line 43/RConn1
  Bus8/LConn1 -- 22mm^2 Line 6/LConn1
  100mm^2 Line 14/LConn2 -- Bus14/RConn2
  Load20/LConn1 -- Bus32/RConn1
  Bus44/LConn1 -- 100mm^2 Line 42/LConn1
  Bus55/LConn1 -- 50mm^2 Line 53/LConn1
  Bus62/LConn1 -- 50mm^2 Line 60/LConn1
  Bus74/LConn2 -- 22mm^2 Line 72/RConn2
  Bus53/LConn1 -- 22mm^2 Line 51/LConn1
  Bus43/LConn3 -- 100mm^2 Line 41/LConn3
  100mm^2 Line 12/RConn3 -- Bus14/LConn3
  Bus25/LConn2 -- 100mm^2 Line 23/RConn2
  Bus64/RConn2 -- Load41/LConn2
  Bus46/LConn3 -- 100mm^2 Line 44/LConn3
  Bus71/RConn1 -- Load46/LConn1
  Load27/LConn1 -- Bus41/RConn1
  Bus31/LConn4 -- 100mm^2 Line 29/RConn4
  22mm^2 Line 5/RConn1 -- Bus7/LConn1
  Bus62/LConn2 -- 50mm^2 Line 60/LConn2
  Bus5/LConn3 -- XLPE 185/90 Line 3/RConn3
  Bus39/LConn3 -- 100mm^2 Line 37/LConn3
  Bus74/RConn4 -- Load49/LConn4
  Bus53/RConn1 -- Load34/LConn1
  22mm^2 Line 70/LConn1 -- Bus72/LConn1
  Bus44/LConn3 -- 100mm^2 Line 42/LConn3
  Bus44/LConn2 -- 100mm^2 Line 42/LConn2
  Bus70/LConn2 -- 100mm^2 Line 68/RConn2
  Bus43/LConn2 -- 100mm^2 Line 41/LConn2
  Bus52/LConn4 -- 100mm^2 Line 50/LConn4
  Bus32/RConn2 -- Load20/LConn2
  Bus41/LConn2 -- 22mm^2 Line 39/LConn2
  Bus53/RConn2 -- Load34/LConn2
  100mm^2 Line 7/RConn2 -- Bus9/LConn2
  Bus2/RConn1 -- XLPE 185/90 Line 1/LConn1
  100mm^2 Line 28/RConn2 -- Bus30/LConn2
  100mm^2 Line 28/RConn3 -- Bus30/LConn3
  Bus47/RConn1 -- Load30/LConn1
  Bus50/LConn4 -- 22mm^2 Line 48/RConn4
  Bus45/LConn3 -- 22mm^2 Line 43/RConn3
  Bus17/LConn1 -- 22mm^2 Line 15/LConn1
  Bus46/LConn1 -- 100mm^2 Line 44/LConn1
  Bus20/LConn2 -- 100mm^2 Line 18/RConn2
  Bus19/LConn2 -- 22mm^2 Line 17/RConn2
  Bus65/RConn1 -- Load42/LConn1
  Bus36/LConn1 -- 16mm^2 Line 34/RConn1
  Bus6/RConn2 -- Load2/LConn2
  22mm^2 Line 27/RConn1 -- Bus29/LConn1
  Bus18/RConn1 -- Load11/LConn1
  16mm^2 Line 8/RConn2 -- Bus10/LConn2
  Bus20/LConn3 -- 100mm^2 Line 18/RConn3
  100mm^2 Line 20/LConn1 -- Bus20/RConn1
  Load26/LConn4 -- Bus40/RConn4
  Bus46/LConn2 -- 100mm^2 Line 44/LConn2
  Load19/LConn2 -- Bus29/RConn2
  Bus2/LConn1 -- Bus1/RConn1
  Bus1/RConn2 -- Bus2/LConn2
  Bus1/RConn3 -- Bus2/LConn3
